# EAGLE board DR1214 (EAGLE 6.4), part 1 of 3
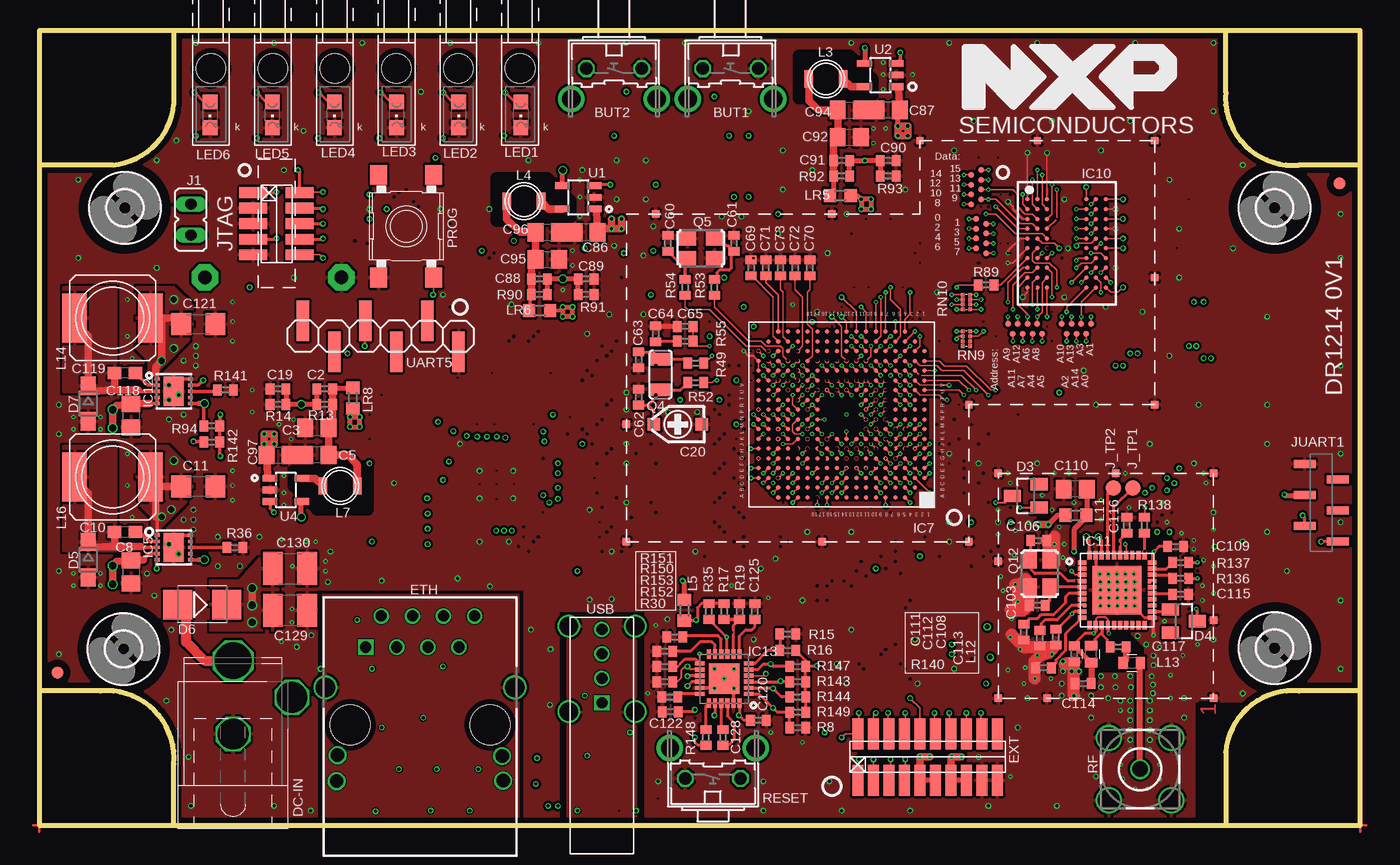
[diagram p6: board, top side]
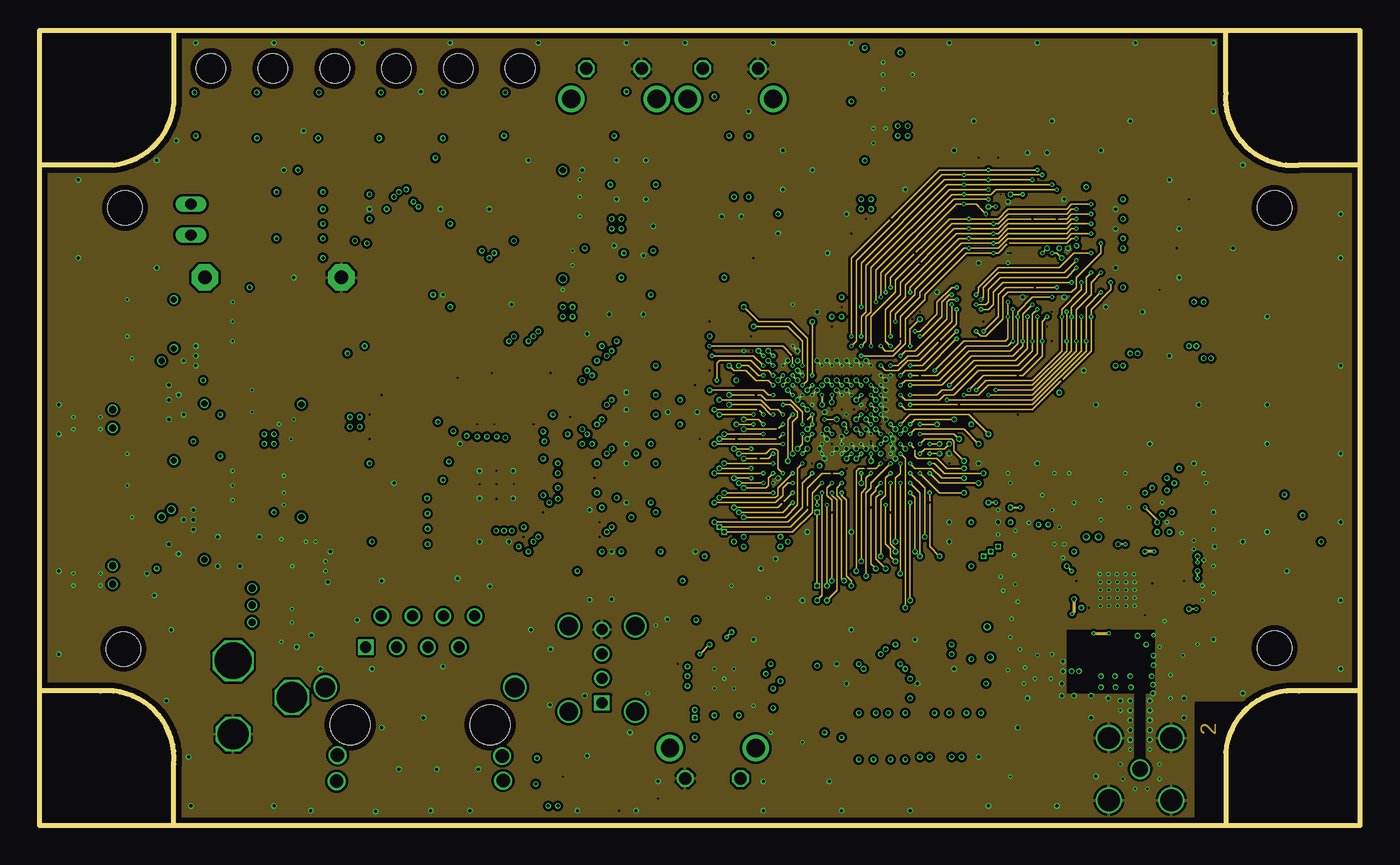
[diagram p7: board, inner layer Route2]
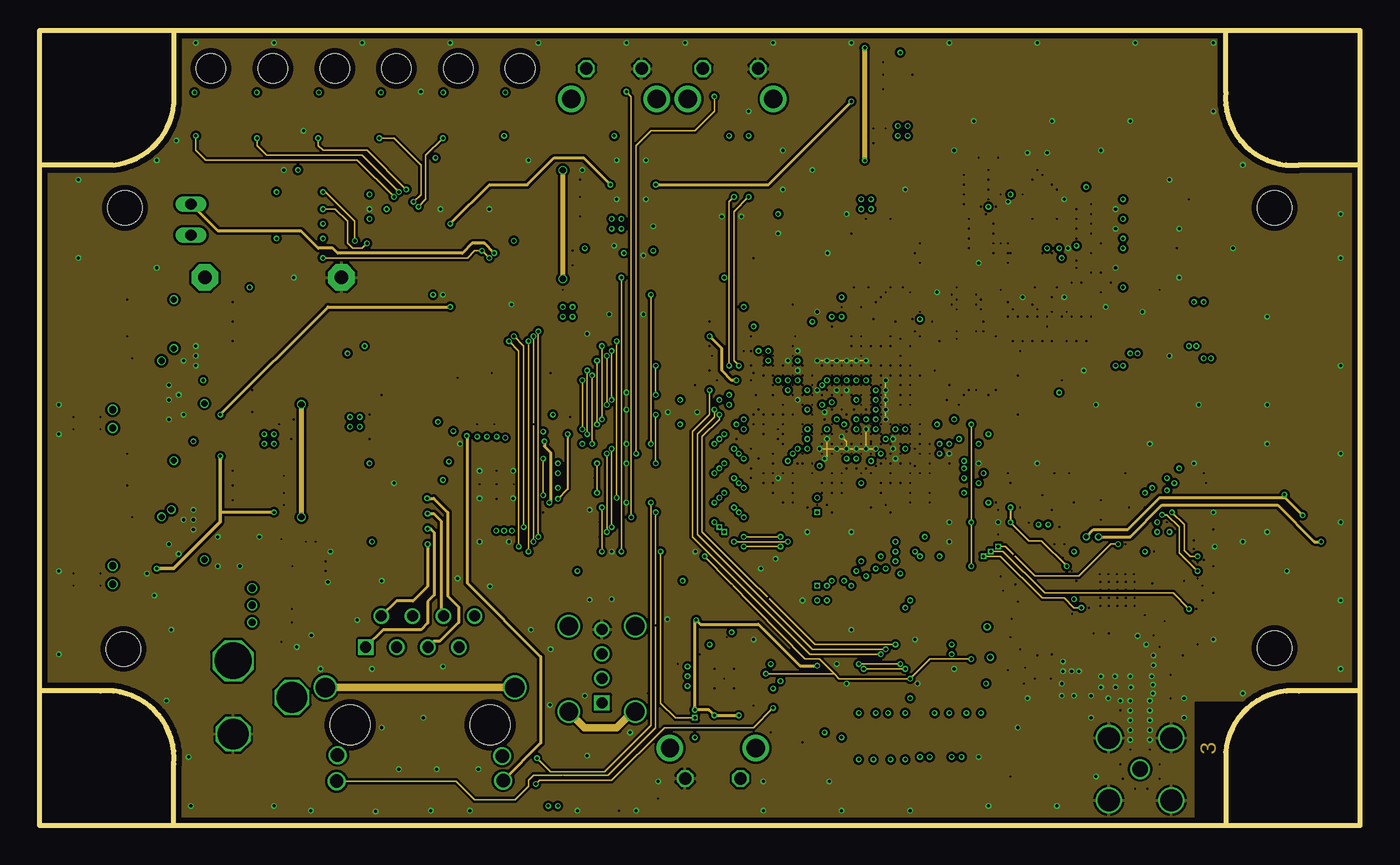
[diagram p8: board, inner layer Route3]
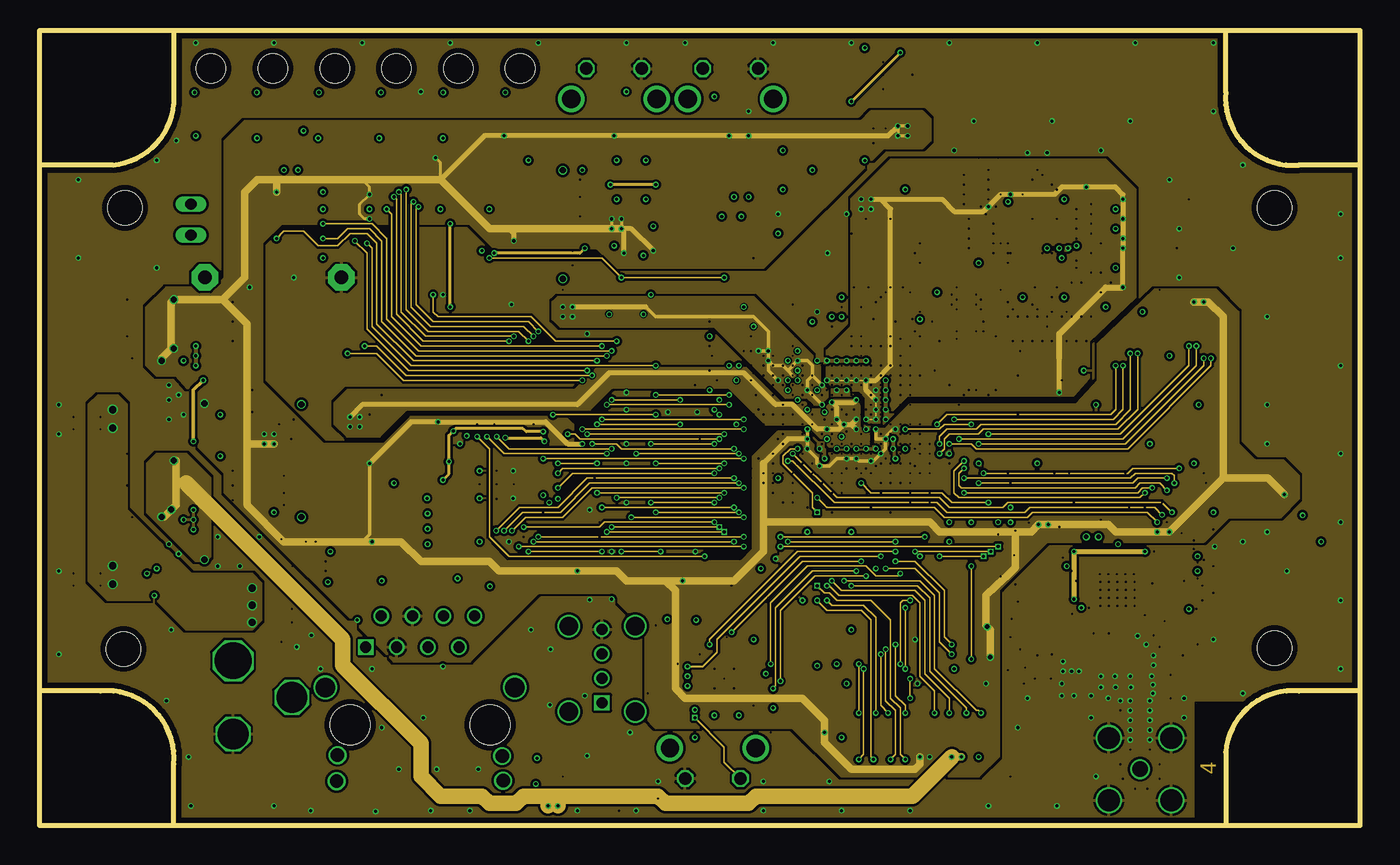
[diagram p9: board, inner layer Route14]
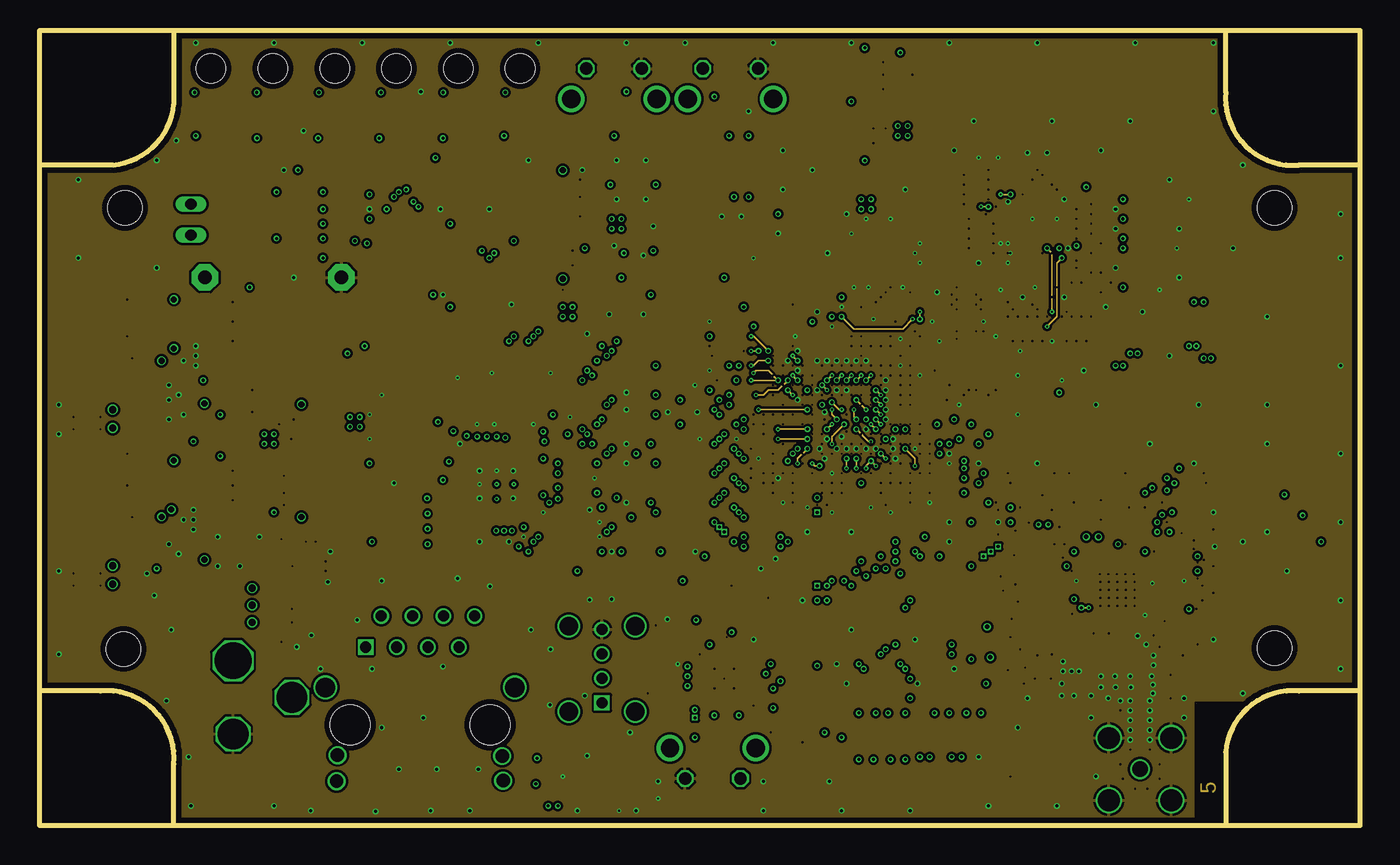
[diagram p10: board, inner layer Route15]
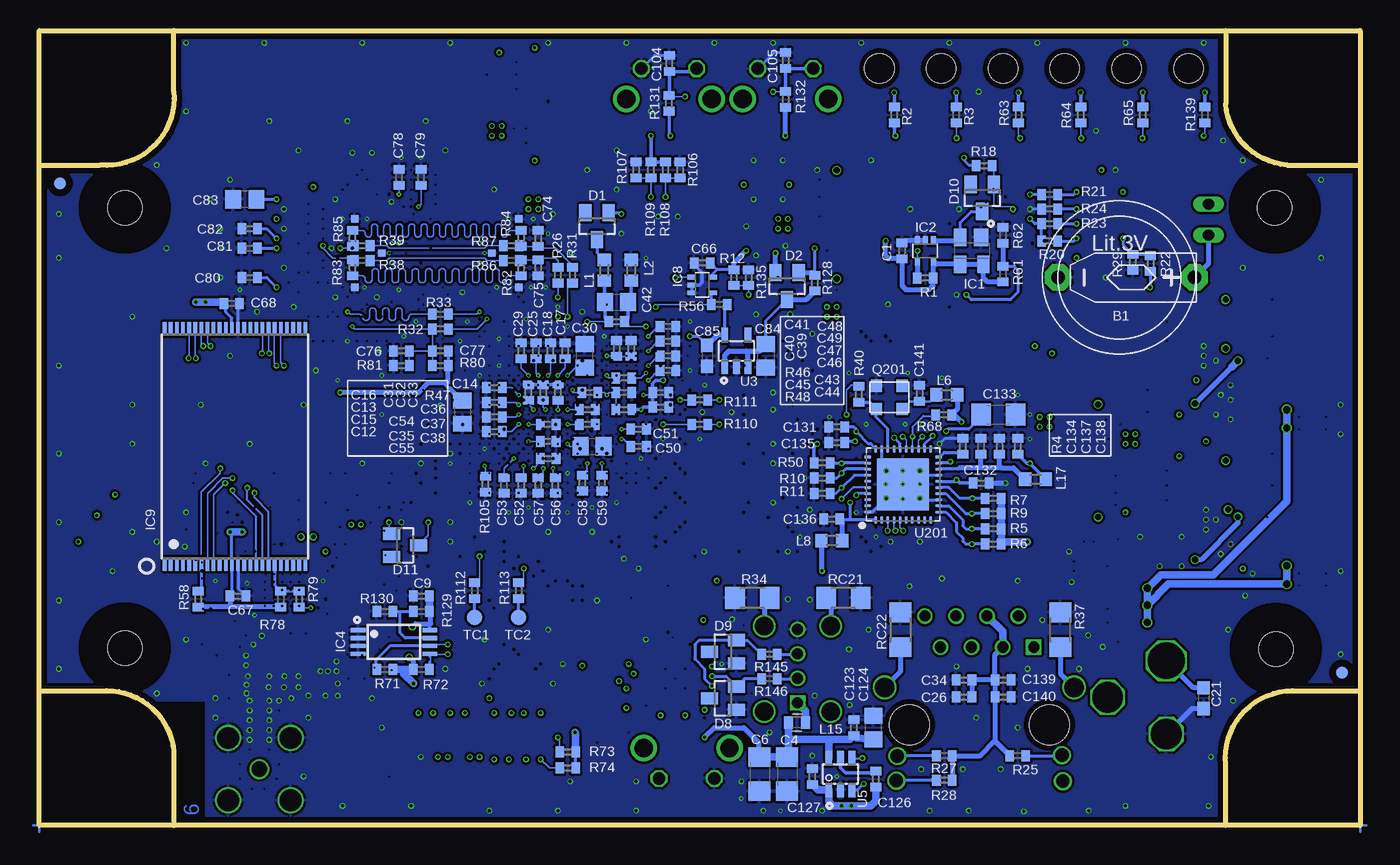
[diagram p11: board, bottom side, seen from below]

Size 108 x 65 mm. Coordinates in mm from the lower left corner, seen from the top.
Outline: 108,0 108,65
Outline: 108,65 0,65
Outline: 11,0 97,0
Outline: 97,0 108,0
Outline: 108,0 108,11
Outline: 108,11 108,54
Outline: 108,54 108,65
Outline: 108,65 97,65
Outline: 97,65 11,65
Outline: 11,65 0,65
Outline: 0,65 0,54
Outline: 0,54 0,11
Outline: 0,11 0,0 11,0
Outline: 11,0 11,5 arc100 5,11 0,11
Outline: 11,65 11,59 arc-80 6,54 0,54
Outline: 108,54 103,54 arc-100 97,60 97,65
Outline: 108,11 103,11 arc90 97,6 97,0
Copper layers ([2:1+(2*3+14*15)+16:15]): Top 0.012mm / dielectric 0.15mm / Route2 0.018mm / dielectric 0.3mm / Route3 0.018mm / dielectric 0.3mm / Route14 0.018mm / dielectric 0.3mm / Route15 0.018mm / dielectric 0.15mm / Bottom 0.012mm
Design rules "eC-TECH_pool-6-layer *": minimum track width 0.1mm, minimum drill 0.15mm, track to track 0.1mm, track to pad 0.1mm, pad to pad 0.1mm, via to via 0.1mm, smd to smd 0.1mm, copper to edge 0.45mm, drill to drill 0.3mm, minimum pad ring 0.175mm, minimum via ring 0.1mm, stop-mask expansion 0.1mm, vias tented up to drill 0.15mm, thermal gap 0.2mm
Net classes: 1 high_pow: width 1.27 mm; 2 med_pow: width 0.61 mm
tRestrict: area 37.4,49.5 to 43.4,52.9; area 20.8,25.9 to 26.8,29.3; area 62.1,59.5 to 68.1,62.9; area 58.8,26.8 to 72.4,40.4; area 85.6,12 to 90,16.9; area 80.8,44 to 82.4,51.2; area 85.6,44 to 87.2,51.2

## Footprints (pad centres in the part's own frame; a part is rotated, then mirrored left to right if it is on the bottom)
B0,5MM = smd 0.5 x 0.5: TP 0,0
CR1225H = drill 1.1 pad 2.184 octagon: + 0,6.16; - 0,-5
TACT90L = drill 1.016 octagon: 1 -2.261,-1.245; 2 2.261,-1.245 | drill 1.499 pad 2.159: 3 -3.505,1.245; 4 3.505,1.245
C0402 = smd 0.7 x 0.9: 1 -0.65,0; 2 0.65,0
C0805 = smd 1.3 x 1.5: 1 -0.95,0; 2 0.95,0
C1206 = smd 1.6 x 1.8: 1 -1.4,0; 2 1.4,0
C0603 = smd 1.1 x 1: 1 -0.85,0; 2 0.85,0
CTRIMCTZ3 = smd 1.016 x 1.016: 1 0,1.95; 2 0,-1.95
C1210 = smd 1.6 x 2.7: 1 -1.4,0; 2 1.4,0
SOT23 = smd 1 x 1.4: 1 -0.95,-1.1; 2 0.95,-1.1; 3 0,1.1
SOD323-W = smd 1.5 x 1.2: A 1.45,0; C -1.45,0
SOD128 = smd 2.4 x 2.4: A 2,0; C -2,0
DC_BIGHOLES = drill 2.5 octagon: 1 -3,0; 2 0,-4.8 | drill 3 octagon: 3 3,0
MODULARJACK8_L = drill 0.9 square: 1 -4.445,6.35 | drill 0.9: 2 -3.175,8.89; 3 -1.905,6.35; 4 -0.635,8.89; 5 0.635,6.35; 6 1.905,8.89; 7 3.175,6.35; 8 4.445,8.89 | drill 1.1: A1 -6.752,-2.491; A2 6.705,-2.561; C1 -6.828,-4.619; C2 6.781,-4.574 | drill 1.6: S1 -7.745,3.05; S2 7.745,3.05 | hole 3.25: -5.715,0; 5.715,0
127_2R20_SMT = smd 0.889 x 2.54: 1 -5.08,-1.905; 2 -5.08,1.905; 3 -3.81,-1.905; 4 -3.81,1.905; 5 -2.54,-1.905; 6 -2.54,1.905; 7 -1.27,-1.905; 8 -1.27,1.905; 9 0,-1.905; 10 0,1.905; 11 1.27,-1.905; 12 1.27,1.905; 13 2.54,-1.905; 14 2.54,1.905; 15 3.81,-1.905; 16 3.81,1.905; 17 5.08,-1.905; 18 5.08,1.905; 19 6.35,-1.905; 20 6.35,1.905
2,8 = hole 2.8: 0,0
SOT143 = smd 1.2 x 1.44: 1 -0.75,-1.1 | smd 1 x 1.44: 2 0.95,-1.1; 3 0.95,1.1; 4 -0.95,1.1
SC70-5 = smd 0.4 x 0.7: 1 -0.65,-0.85; 2 0,-0.85; 3 0.65,-0.85; 4 0.65,0.85; 5 -0.65,0.85
TSSOP8 = smd 0.35 x 1.2: 1 -0.975,-2.925; 2 -0.325,-2.925; 3 0.325,-2.925; 4 0.975,-2.925; 5 0.975,2.925; 6 0.325,2.925; 7 -0.325,2.925; 8 -0.975,2.925
DFN10-3X3 = smd 0.25 x 0.45: 1 -1,-1.35; 2 -0.5,-1.35; 3 0,-1.35; 4 0.5,-1.35; 5 1,-1.35; 6 1,1.35; 7 0.5,1.35; 8 0,1.35; 9 -0.5,1.35; 10 -1,1.35 | smd 2.38 x 1.65: EXP 0,0
SOT1048-1 = smd 0.35 x 0.35: A3 -5.184,6.779; A4 -4.387,6.779; A5 -3.589,6.779; A6 -2.792,6.779; A7 -1.994,6.779; A8 -1.196,6.779; A9 -0.399,6.779; A10 0.399,6.779; A11 1.196,6.779; A12 1.994,6.779; A13 2.791,6.779; A14 3.589,6.779; A15 4.386,6.779; A16 5.184,6.779; B2 -5.982,5.982; B3 -5.184,5.982; B4 -4.387,5.982; B5 -3.589,5.982; B6 -2.792,5.982; B7 -1.994,5.982; B8 -1.196,5.982; B9 -0.399,5.982; B10 0.399,5.982; B11 1.196,5.982; B12 1.994,5.982; B13 2.791,5.982; B14 3.589,5.982; B15 4.386,5.982; B16 5.184,5.982; B17 5.982,5.982; C1 -6.779,5.184; C2 -5.982,5.184; C3 -5.184,5.184; C4 -4.387,5.184; C5 -3.589,5.184; C6 -2.792,5.184; C7 -1.994,5.184; C8 -1.196,5.184; C9 -0.399,5.184; C10 0.399,5.184; C11 1.196,5.184; C12 1.994,5.184; C13 2.791,5.184; C14 3.589,5.184; C15 4.386,5.184; C16 5.184,5.184; C17 5.982,5.184; C18 6.779,5.184; D1 -6.779,4.387; D2 -5.982,4.387; D3 -5.184,4.387; D4 -4.387,4.387; D5 -3.589,4.387; D6 -2.792,4.387; D7 -1.994,4.387; D8 -1.196,4.387; D9 -0.399,4.387; D10 0.399,4.387; D11 1.196,4.387; D12 1.994,4.387; D13 2.791,4.387; D14 3.589,4.387; D15 4.386,4.387; D16 5.184,4.387; D17 5.982,4.387; D18 6.779,4.387; E1 -6.779,3.589; E2 -5.982,3.589; E3 -5.184,3.589; E4 -4.387,3.589; E5 -3.589,3.589; E6 -2.792,3.589; E7 -1.994,3.589; E8 -1.196,3.589; E9 -0.399,3.589; E10 0.399,3.589; E11 1.196,3.589; E12 1.994,3.589; E13 2.791,3.589; E14 3.589,3.589; E15 4.386,3.589; E16 5.184,3.589; E17 5.982,3.589; E18 6.779,3.589; F1 -6.779,2.792; F2 -5.982,2.792; F3 -5.184,2.792; F4 -4.387,2.792; F5 -3.589,2.792; F6 -2.792,2.792; F7 -1.994,2.792; F8 -1.196,2.792; F9 -0.399,2.792; F10 0.399,2.792; F11 1.196,2.792; F12 1.994,2.792; F13 2.791,2.792; F14 3.589,2.792; F15 4.386,2.792; F16 5.184,2.792; F17 5.982,2.792; F18 6.779,2.792; G1 -6.779,1.994; G2 -5.982,1.994; G3 -5.184,1.994; G4 -4.387,1.994; G5 -3.589,1.994; G6 -2.792,1.994; G7 -1.994,1.994; G8 -1.196,1.994; G9 -0.399,1.994; G10 0.399,1.994; G11 1.196,1.994; G12 1.994,1.994; G13 2.791,1.994; G14 3.589,1.994; G15 4.386,1.994; G16 5.184,1.994; G17 5.982,1.994; G18 6.779,1.994; H1 -6.779,1.196; H2 -5.982,1.196; H3 -5.184,1.196; H4 -4.387,1.196; H5 -3.589,1.196; H6 -2.792,1.196; H7 -1.994,1.196; H12 1.994,1.196; H13 2.791,1.196; H14 3.589,1.196; H15 4.386,1.196; H16 5.184,1.196; H17 5.982,1.196; H18 6.779,1.196; J1 -6.779,0.399; J2 -5.982,0.399; J3 -5.184,0.399; J4 -4.387,0.399; J5 -3.589,0.399; J6 -2.792,0.399; J7 -1.994,0.399; J12 1.994,0.399; J13 2.791,0.399; J14 3.589,0.399; J15 4.386,0.399; J16 5.184,0.399; J17 5.982,0.399; J18 6.779,0.399; K1 -6.779,-0.399; K2 -5.982,-0.399; K3 -5.184,-0.399; K4 -4.387,-0.399; K5 -3.589,-0.399; K6 -2.792,-0.399; K7 -1.994,-0.399; K12 1.994,-0.399; K13 2.791,-0.399; K14 3.589,-0.399; K15 4.386,-0.399; K16 5.184,-0.399; K17 5.982,-0.399; K18 6.779,-0.399; L1 -6.779,-1.196; L2 -5.982,-1.196; L3 -5.184,-1.196; L4 -4.387,-1.196; L5 -3.589,-1.196; L6 -2.792,-1.196; L7 -1.994,-1.196; L12 1.994,-1.196; L13 2.791,-1.196; L14 3.589,-1.196; L15 4.386,-1.196; L16 5.184,-1.196; L17 5.982,-1.196; L18 6.779,-1.196; M1 -6.779,-1.994; M2 -5.982,-1.994; M3 -5.184,-1.994; M4 -4.387,-1.994; M5 -3.589,-1.994; M6 -2.792,-1.994; M7 -1.994,-1.994; M8 -1.196,-1.994; M9 -0.399,-1.994; M10 0.399,-1.994; M11 1.196,-1.994; M12 1.994,-1.994; M13 2.791,-1.994; M14 3.589,-1.994; M15 4.386,-1.994; M16 5.184,-1.994; M17 5.982,-1.994; M18 6.779,-1.994; N1 -6.779,-2.791; N2 -5.982,-2.791; N3 -5.184,-2.791; N4 -4.387,-2.791; N5 -3.589,-2.791; N6 -2.792,-2.791; N7 -1.994,-2.791; N8 -1.196,-2.791; N9 -0.399,-2.791; N10 0.399,-2.791; N11 1.196,-2.791; N12 1.994,-2.791; N13 2.791,-2.791; N14 3.589,-2.791; N15 4.386,-2.791; N16 5.184,-2.791; N17 5.982,-2.791; N18 6.779,-2.791; P1 -6.779,-3.589; P2 -5.982,-3.589; P3 -5.184,-3.589; P4 -4.387,-3.589; P5 -3.589,-3.589; P6 -2.792,-3.589; P7 -1.994,-3.589; P8 -1.196,-3.589; P9 -0.399,-3.589; P10 0.399,-3.589; P11 1.196,-3.589; P12 1.994,-3.589; P13 2.791,-3.589; P14 3.589,-3.589; P15 4.386,-3.589; P16 5.184,-3.589; P17 5.982,-3.589; P18 6.779,-3.589; R1 -6.779,-4.386; R2 -5.982,-4.386; R3 -5.184,-4.386; R4 -4.387,-4.386; R5 -3.589,-4.386; R6 -2.792,-4.386; R7 -1.994,-4.386; R8 -1.196,-4.386; R9 -0.399,-4.386; R10 0.399,-4.386; R11 1.196,-4.386; R12 1.994,-4.386; R13 2.791,-4.386; R14 3.589,-4.386; R15 4.386,-4.386; R16 5.184,-4.386; R17 5.982,-4.386; R18 6.779,-4.386; T1 -6.779,-5.184; T2 -5.982,-5.184; T3 -5.184,-5.184; T4 -4.387,-5.184; T5 -3.589,-5.184; T6 -2.792,-5.184; T7 -1.994,-5.184; T8 -1.196,-5.184; T9 -0.399,-5.184; T10 0.399,-5.184; T11 1.196,-5.184; T12 1.994,-5.184; T13 2.791,-5.184; T14 3.589,-5.184; T15 4.386,-5.184; T16 5.184,-5.184; T17 5.982,-5.184; T18 6.779,-5.184; U2 -5.982,-5.982; U3 -5.184,-5.982; U4 -4.387,-5.982; U5 -3.589,-5.982; U6 -2.792,-5.982; U7 -1.994,-5.982; U8 -1.196,-5.982; U9 -0.399,-5.982; U10 0.399,-5.982; U11 1.196,-5.982; U12 1.994,-5.982; U13 2.791,-5.982; U14 3.589,-5.982; U15 4.386,-5.982; U16 5.184,-5.982; U17 5.982,-5.982; V3 -5.184,-6.779; V4 -4.387,-6.779; V5 -3.589,-6.779; V6 -2.792,-6.779; V7 -1.994,-6.779; V8 -1.196,-6.779; V9 -0.399,-6.779; V10 0.399,-6.779; V11 1.196,-6.779; V12 1.994,-6.779; V13 2.791,-6.779; V14 3.589,-6.779; V15 4.386,-6.779; V16 5.184,-6.779
TSOP48 = smd 1.1 x 0.3: 1 -9.625,5.75; 2 -9.625,5.25; 3 -9.625,4.75; 4 -9.625,4.25; 5 -9.625,3.75; 6 -9.625,3.25; 7 -9.625,2.75; 8 -9.625,2.25; 9 -9.625,1.75; 10 -9.625,1.25; 11 -9.625,0.75; 12 -9.625,0.25; 13 -9.625,-0.25; 14 -9.625,-0.75; 15 -9.625,-1.25; 16 -9.625,-1.75; 17 -9.625,-2.25; 18 -9.625,-2.75; 19 -9.625,-3.25; 20 -9.625,-3.75; 21 -9.625,-4.25; 22 -9.625,-4.75; 23 -9.625,-5.25; 24 -9.625,-5.75; 25 9.625,-5.75; 26 9.625,-5.25; 27 9.625,-4.75; 28 9.625,-4.25; 29 9.625,-3.75; 30 9.625,-3.25; 31 9.625,-2.75; 32 9.625,-2.25; 33 9.625,-1.75; 34 9.625,-1.25; 35 9.625,-0.75; 36 9.625,-0.25; 37 9.625,0.25; 38 9.625,0.75; 39 9.625,1.25; 40 9.625,1.75; 41 9.625,2.25; 42 9.625,2.75; 43 9.625,3.25; 44 9.625,3.75; 45 9.625,4.25; 46 9.625,4.75; 47 9.625,5.25; 48 9.625,5.75
FBGA60-6X10 = smd 0.35 x 0.35: A1 -3.2,3.6; A2 -2.4,3.6; A3 -1.6,3.6; A7 1.6,3.6; A8 2.4,3.6; A9 3.2,3.6; B1 -3.2,2.8; B2 -2.4,2.8; B3 -1.6,2.8; B7 1.6,2.8; B8 2.4,2.8; B9 3.2,2.8; C1 -3.2,2; C2 -2.4,2; C3 -1.6,2; C7 1.6,2; C8 2.4,2; C9 3.2,2; D1 -3.2,1.2; D2 -2.4,1.2; D3 -1.6,1.2; D7 1.6,1.2; D8 2.4,1.2; D9 3.2,1.2; E1 -3.2,0.4; E2 -2.4,0.4; E3 -1.6,0.4; E7 1.6,0.4; E8 2.4,0.4; E9 3.2,0.4; F1 -3.2,-0.4; F2 -2.4,-0.4; F3 -1.6,-0.4; F7 1.6,-0.4; F8 2.4,-0.4; F9 3.2,-0.4; G1 -3.2,-1.2; G2 -2.4,-1.2; G3 -1.6,-1.2; G7 1.6,-1.2; G8 2.4,-1.2; G9 3.2,-1.2; H1 -3.2,-2; H2 -2.4,-2; H3 -1.6,-2; H7 1.6,-2; H8 2.4,-2; H9 3.2,-2; J1 -3.2,-2.8; J2 -2.4,-2.8; J3 -1.6,-2.8; J7 1.6,-2.8; J8 2.4,-2.8; J9 3.2,-2.8; K1 -3.2,-3.6; K2 -2.4,-3.6; K3 -1.6,-3.6; K7 1.6,-3.6; K8 2.4,-3.6; K9 3.2,-3.6
SOT618-1 = smd 0.7 x 0.36: 1 -2.875,2.25; 2 -2.875,1.75; 3 -2.875,1.25; 4 -2.875,0.75; 5 -2.875,0.25; 6 -2.875,-0.25; 7 -2.875,-0.75; 8 -2.875,-1.25; 9 -2.875,-1.75; 10 -2.875,-2.25; 21 2.875,-2.25; 22 2.875,-1.75; 23 2.875,-1.25; 24 2.875,-0.75; 25 2.875,-0.25; 26 2.875,0.25; 27 2.875,0.75; 28 2.875,1.25; 29 2.875,1.75; 30 2.875,2.25 | smd 0.36 x 0.7: 11 -2.25,-2.875; 12 -1.75,-2.875; 13 -1.25,-2.875; 14 -0.75,-2.875; 15 -0.25,-2.875; 16 0.25,-2.875; 17 0.75,-2.875; 18 1.25,-2.875; 19 1.75,-2.875; 20 2.25,-2.875; 31 2.25,2.875; 32 1.75,2.875; 33 1.25,2.875; 34 0.75,2.875; 35 0.25,2.875; 36 -0.25,2.875; 37 -0.75,2.875; 38 -1.25,2.875; 39 -1.75,2.875; 40 -2.25,2.875 | smd 4 x 4: VSSA 0,0
HVQFN24-4X4 = smd 0.8 x 0.35: 1 -2,1.25; 2 -2,0.75; 3 -2,0.25; 4 -2,-0.25; 5 -2,-0.75; 6 -2,-1.25; 13 2,-1.25; 14 2,-0.75; 15 2,-0.25; 16 2,0.25; 17 2,0.75; 18 2,1.25 | smd 0.35 x 0.8: 7 -1.25,-2; 8 -0.75,-2; 9 -0.25,-2; 10 0.25,-2; 11 0.75,-2; 12 1.25,-2; 19 1.25,2; 20 0.75,2; 21 0.25,2; 22 -0.25,2; 23 -0.75,2; 24 -1.25,2 | smd 2.5 x 2.5: GND 0,0
JP1 = drill 0.914 long: 1 0,-1.27; 2 0,1.27
B1,27 = smd 1.27 x 1.27: TP 0,0
127_2R10_SMT = smd 0.889 x 2.286: 1 -2.54,-1.905; 2 -2.54,1.905; 3 -1.27,-1.905; 4 -1.27,1.905; 5 0,-1.905; 6 0,1.905; 7 1.27,-1.905; 8 1.27,1.905; 9 2.54,-1.905; 10 2.54,1.905
BD075-06-A-1-L-D = smd 0.65 x 1.8: 1 -3.175,-1.35; 2 -1.905,1.35; 3 -0.635,-1.35; 4 0.635,1.35; 5 1.905,-1.35; 6 3.175,1.35
R0603 = smd 1 x 1.1: 1 -0.85,0; 2 0.85,0
COIL2.8MM = smd 0.7 x 1.4: P$1 -1.4,0; P$2 1.4,0
PACKAGE0603 = smd 1 x 1.1: 1 -0.85,0; 2 0.85,0
P0603 = smd 0.762 x 1.016: 1 -0.7,0; 2 0.7,0
COIL7070 = smd 4 x 2: 1 0,3.104; 2 0,-3.104
CHIPLED_0805 = smd 1.2 x 1.2: A 0,-1.05; C 0,1.05
B3XS = smd 1.6 x 1.4: 1 -4.2,2.25; 2 4.2,2.25; 3 -4.2,-2.25; 4 4.2,-2.25
XTAL2 = smd 1 x 1.8: 1 -1.19,0; 2 1.31,0
XTAL4 = smd 1.4 x 1.15: 1 -1.6,-0.8; 2 0.6,-0.8; 3 0.6,0.8; 4 -1.6,0.8
ASE = smd 0.9 x 1: 1 -1.05,-0.95; 3 1.05,-0.95; 4 1.05,0.95; 6 -1.05,0.95
R0402 = smd 0.7 x 0.9: 1 -0.65,0; 2 0.65,0
R1206 = smd 1.6 x 1.803: 1 -1.422,0; 2 1.422,0
TACT90 = drill 1.016 octagon: 1 -2.261,0.025; 2 2.261,0.025 | drill 1.499 pad 2.159: 3 -3.505,2.515; 4 3.505,2.515
BU-SMA-V = drill 1.27: 1 0,0 | drill 1.778: 2 -2.55,2.55; 3 2.55,2.55; 4 2.55,-2.55; 5 -2.55,-2.55
EXB18V = smd 0.3 x 0.3: 1 -0.6,-0.3; 2 -0.2,-0.3; 3 0.2,-0.3; 4 0.6,-0.3; 5 0.6,0.3; 6 0.2,0.3; 7 -0.2,0.3; 8 -0.6,0.3
TP06SQ = smd 0.6 x 0.6: TP 0,0
SOT23-5 = smd 0.55 x 1.2: 1 -0.95,-1.3; 2 0,-1.3; 3 0.95,-1.3; 4 0.95,1.3; 5 -0.95,1.3
SOT23-6 = smd 0.55 x 1.2: 1 -0.95,-1.3; 2 0,-1.3; 3 0.95,-1.3; 4 0.95,1.3; 5 0,1.3; 6 -0.95,1.3
MVER_ETHERNET_LLP40 = smd 0.25 x 0.6: 1 2.25,2.9; 2 1.75,2.9; 3 1.25,2.9; 4 0.75,2.9; 5 0.25,2.9; 6 -0.25,2.9; 7 -0.75,2.9; 8 -1.25,2.9; 9 -1.75,2.9; 10 -2.25,2.9; 21 -2.25,-2.9; 22 -1.75,-2.9; 23 -1.25,-2.9; 24 -0.75,-2.9; 25 -0.25,-2.9; 26 0.25,-2.9; 27 0.75,-2.9; 28 1.25,-2.9; 29 1.75,-2.9; 30 2.25,-2.9 | smd 0.6 x 0.25: 11 -2.9,2.25; 12 -2.9,1.75; 13 -2.9,1.25; 14 -2.9,0.75; 15 -2.9,0.25; 16 -2.9,-0.25; 17 -2.9,-0.75; 18 -2.9,-1.25; 19 -2.9,-1.75; 20 -2.9,-2.25; 31 2.9,-2.25; 32 2.9,-1.75; 33 2.9,-1.25; 34 2.9,-0.75; 35 2.9,-0.25; 36 2.9,0.25; 37 2.9,0.75; 38 2.9,1.25; 39 2.9,1.75; 40 2.9,2.25 | smd 4.3 x 4.3: 41 0,0
LIGHTPIPE6 = hole 2.4: -12.64,0; -7.59,0; -2.54,0; 2.51,0; 7.56,0; 12.64,0
FIDUCIAL_1MMCIRCLE = smd 1 x 1: P$1 0,0
1X06SMD = smd 1.016 x 3.302: 1 -1.27,1.27; 2 1.27,-1.27; 3 3.81,1.27; 4 6.35,-1.27; 5 8.89,1.27; 6 11.43,-1.27
USB_A_HU = drill 0.9 square: 1 0.73,0 | drill 0.9: 2 2.73,0; 3 4.73,0; 4 6.73,0 | drill 1.5: P$5 0,2.72; P$6 0,-2.72; P$7 7,2.72; P$8 7,-2.72

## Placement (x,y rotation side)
0  TP0.5  [B0,5MM]  76.6,49.6 0 top
1  TP0.5  [B0,5MM]  77.4,49.2 0 top
2  TP0.5  [B0,5MM]  76.6,48.8 0 top
3  TP0.5  [B0,5MM]  77.4,48.4 0 top
4  TP0.5  [B0,5MM]  76.6,48 0 top
5  TP0.5  [B0,5MM]  77.4,47.6 0 top
6  TP0.5  [B0,5MM]  76.6,47.2 0 top
7  TP0.5  [B0,5MM]  77.4,46.8 0 top
8  TP0.5  [B0,5MM]  76.2,50.8 0 top
9  TP0.5  [B0,5MM]  77,51.2 0 top
10  TP0.5  [B0,5MM]  76.2,51.6 0 top
11  TP0.5  [B0,5MM]  77,52 0 top
12  TP0.5  [B0,5MM]  76.2,52.4 0 top
13  TP0.5  [B0,5MM]  77,52.8 0 top
14  TP0.5  [B0,5MM]  76.2,53.2 0 top
15  TP0.5  [B0,5MM]  77,53.6 0 top
A0  TP0.5  [B0,5MM]  85.6,40.2 0 top
A1  TP0.5  [B0,5MM]  86,41 0 top
A2  TP0.5  [B0,5MM]  84,40.2 0 top
A3  TP0.5  [B0,5MM]  85.2,41 0 top
A4  TP0.5  [B0,5MM]  81.2,40.2 0 top
A5  TP0.5  [B0,5MM]  82,40.2 0 top
A6  TP0.5  [B0,5MM]  80.8,41 0 top
A7  TP0.5  [B0,5MM]  80.4,40.2 0 top
A8  TP0.5  [B0,5MM]  81.6,41 0 top
A9  TP0.5  [B0,5MM]  79.2,41 0 top
A10  TP0.5  [B0,5MM]  83.6,41 0 top
A11  TP0.5  [B0,5MM]  79.6,40.2 0 top
A12  TP0.5  [B0,5MM]  80,41 0 top
A13  TP0.5  [B0,5MM]  84.4,41 0 top
A14  TP0.5  [B0,5MM]  84.8,40.2 0 top
B1  CR1225H  [CR1225H]  19.7,44.81 270 bottom
BUT1  MCDTSA6-5K  [TACT90L]  56.52,60.64 180 top
BUT2  MCDTSA6-5K  [TACT90L]  46.99,60.64 180 top
C1  100n  [C0402]  37.47,46.99 90 bottom
C2  12p  [C0402]  23.34,35.7 180 top
C3  4u7/X7R  [C0805]  22.7,32.52 180 top
C4  22u/X7R  [C1206]  46.85,4.2 270 bottom
C5  4u7/X7R  [C0805]  22.7,30.3 180 top
C6  22u/X7R  [C1206]  49.1,4.2 270 bottom
C8  4u7/X7R  [C0805]  7.5,20.73 270 top
C9  100n  [C0402]  76.75,18.75 0 bottom
C10  470n  [C0603]  7,24 180 top
C11  22u/X7R  [C1206]  13,27.73 0 top
C12  10n  [C0402]  70.8,32.2 180 bottom
C13  100n  [C0402]  70.8,34.6 180 bottom
C14  10u/X7R  [C0805]  73.4,33.8 270 bottom
C15  10n  [C0402]  70.8,33.4 180 bottom
C16  100n  [C0402]  70.8,35.8 180 bottom
C17  10n  [C0402]  65,38.8 90 bottom
C18  10n  [C0402]  66.2,38.8 90 bottom
C19  na  [C0402]  19.52,35.7 180 top
C20  5-20p  [CTRIMCTZ3]  52.2,32.8 90 top
C21  10n/NP0  [C0603]  12.8,10.4 270 bottom
C25  100n  [C0402]  67.4,38.8 90 bottom
C26  100n  [C0402]  32.4,10.5 180 bottom
C29  100n  [C0402]  68.6,38.8 90 bottom
C30  10u/X7R  [C0805]  63.4,38.4 90 bottom
C31  10n  [C0402]  68,35.4 90 bottom
C32  10n  [C0402]  66.8,35.4 90 bottom
C33  10n  [C0402]  65.6,35.4 90 bottom
C34  100n  [C0402]  32.4,11.9 180 bottom
C35  100n  [C0402]  66.4,31.4 0 bottom
C36  100n  [C0402]  63.2,34 0 bottom
C37  100n  [C0402]  63.2,32.8 0 bottom
C38  10u/X7R  [C0805]  62.8,31 0 bottom
C39  10n  [C0402]  59.6,39 90 bottom
C40  100n  [C0402]  60.8,39 90 bottom
C41  10n  [C0402]  60.8,41.2 0 bottom
C42  10u/X7R  [C0805]  60.8,42.8 0 bottom
C43  100n  [C0402]  57.2,35.4 0 bottom
C44  100n  [C0402]  57.2,34.2 0 bottom
C45  100n  [C0402]  60.2,35.4 0 bottom
C46  100n  [C0402]  56.6,37.2 0 bottom
C47  100n  [C0402]  56.6,38.4 0 bottom
C48  100n  [C0402]  56.6,40.8 0 bottom
C49  100n  [C0402]  56.6,39.6 0 bottom
C50  10n  [C0402]  59,31 0 bottom
C51  100n  [C0402]  59,32.4 0 bottom
C52  10n  [C0402]  68.6,27.8 270 bottom
C53  100n  [C0402]  70,27.8 270 bottom
C54  10n  [C0402]  66.4,32.8 0 bottom
C55  100n  [C0402]  66.4,30 0 bottom
C56  10n  [C0402]  65.8,27.8 270 bottom
C57  100n  [C0402]  67.2,27.8 270 bottom
C58  10n  [C0402]  63.6,28 270 bottom
C59  100n  [C0402]  62,28 270 bottom
C60  22p  [C0402]  51.4,47.6 270 top
C61  22p  [C0402]  56.8,47.6 270 top
C62  22p  [C0402]  49,35.03 270 top
C63  22p  [C0402]  49,38.07 90 top
C64  3n9  [C0402]  50.4,40.2 270 top
C65  150p  [C0402]  52.8,40.8 0 top
C66  100n  [C0402]  53.8,46 180 bottom
C67  10n  [C0402]  91.75,18.75 0 bottom
C68  100n  [C0402]  92.27,42.69 0 bottom
C69  1n  [C0402]  58.2,45.6 90 top
C70  1n  [C0402]  63,45.6 90 top
C71  1n  [C0402]  59.4,45.6 90 top
C72  1n  [C0402]  61.8,45.6 90 top
C73  1n  [C0402]  60.6,45.6 90 top
C74  na  [C0402]  67.2,48 90 bottom
C75  na  [C0402]  67.2,45.6 270 bottom
C76  na  [C0402]  78.4,38.8 180 bottom
C77  na  [C0402]  75.2,38.8 180 bottom
C78  10n  [C0402]  78.6,53 90 bottom
C79  10n  [C0402]  76.8,53 90 bottom
C80  100n  [C0402]  90.8,44.8 180 bottom
C81  100n  [C0402]  90.8,47.2 180 bottom
C82  100n  [C0402]  90.8,48.8 180 bottom
C83  10u/X7R  [C0805]  91.2,51.2 180 bottom
C84  4u7/X7R  [C0805]  48.6,38.4 270 bottom
C85  470n/X7R  [C0603]  53.4,38.4 270 bottom
C86  4u7/X7R  [C0805]  44.7,48.5 180 top
C87  4u7/X7R  [C0805]  69.41,58.5 180 top
C88  na  [C0402]  40.9,44.69 0 top
C89  na  [C0402]  44.7,44.69 0 top
C90  na  [C0402]  69.41,54.38 0 top
C91  na  [C0402]  65.59,54.38 0 top
C92  4u7/X7R  [C0805]  66.23,56.28 0 top
C94  4u7/X7R  [C0805]  66.23,58.5 0 top
C95  4u7/X7R  [C0805]  41.53,46.28 0 top
C96  4u7/X7R  [C0805]  41.53,48.5 0 top
C97  4u7/X7R  [C0805]  19.52,30.3 0 top
C103  15p  [C0402]  81.6,18 0 top
C104  22n  [C0402]  56.48,62.3 90 bottom
C105  22n  [C0402]  46.99,62.55 90 bottom
C106  15p  [C0402]  81.7,23.3 180 top
C108  100n/X7R  [C0402]  83.1,15.4 270 top
C109  100n/X7R  [C0402]  92.9,22.8 0 top
C110  10u/X7R  [C0805]  84.7,27.5 180 top
C111  100n/X7R  [C0402]  80.5,15.8 270 top
C112  10n/X7R  [C0402]  81.8,15.3 270 top
C113  47p/NPO  [C0402]  84.62,14.03 270 top
C114  100n/X7R  [C0402]  85.33,11.61 180 top
C115  100n/X7R  [C0402]  93.3,18.9 0 top
C116  100n/X7R  [C0402]  88.9,24.55 90 top
C117  47p/NPO  [C0402]  88.2,14.6 180 top
C118  4u7/X7R  [C0805]  7.5,33.5 270 top
C119  470n  [C0603]  7,37 180 top
C120  100n  [C0402]  58.8,8.6 0 top
C121  22u/X7R  [C1206]  13,41 0 top
C122  100n  [C0402]  51.6,9.3 180 top
C123  100n  [C0402]  41.4,8 90 bottom
C124  4u7/X7R  [C0805]  39.8,8 90 bottom
C125  1u  [C0402]  58.5,17.5 90 top
C126  1n  [C0402]  39.6,3.8 270 bottom
C127  100n  [C0402]  44.8,4 90 bottom
C128  220n  [C0402]  55.9,7.2 270 top
C129  47u/16v  [C1210]  20.5,17.6 0 top
C130  47u/16v  [C1210]  20.5,21 0 top
C131  100n  [C0402]  42.8,32.6 180 bottom
C132  100n  [C0402]  31,28 0 bottom
C133  10u/tantalium  [C1206]  29.59,33.6 0 bottom
C134  1u  [C0402]  31,31 90 bottom
C135  1u  [C0402]  42.8,31.3 180 bottom
C136  100n  [C0402]  43.2,25.05 180 bottom
C137  100n  [C0402]  29.5,31 90 bottom
C138  2u2  [C0402]  28,31 90 bottom
C139  100n  [C0402]  29.2,11.9 0 bottom
C140  100n  [C0402]  29.2,10.5 0 bottom
C141  100n  [C0402]  36.02,35.33 90 bottom
D1  BAT754  [SOT23]  62.4,49 180 bottom
D2  BAT54C  [SOT23]  46.86,44.11 180 bottom
D3  BAT754  [SOT23]  80.65,26.95 90 top
D4  BAT754  [SOT23]  93.58,16.71 270 top
D5  PMEG2010AEJ  [SOD323-W]  4,21.73 270 top
D6  PMEG3020EP  [SOD128]  13.32,18.07 180 top
D7  PMEG2010AEJ  [SOD323-W]  4,34.5 270 top
D8  MMBZ9V1AL  [SOT23]  52.1,10.4 90 bottom
D9  MMBZ9V1AL  [SOT23]  52.1,14.2 90 bottom
D10  BAT754  [SOT23]  30.9,51.32 180 bottom
D11  BAT754  [SOT23]  78.1,22.9 270 bottom
DC-IN  DC10B  [DC_BIGHOLES]  15.85,10.47 90 top
ETH  TE CONNECTIVITY - 5-6605758-1  [MODULARJACK8_L]  31.14,8.23 0 top
EXT  M50-3601042  [127_2R20_SMT]  72,5.6 0 top
FM1  CROSSHAIR8MIL  [CROSSHAIR_8MIL]  108,0 0 top
FM2  CROSSHAIR8MIL  [CROSSHAIR_8MIL]  0,0 0 top
FM3  CROSSHAIR8MIL  [CROSSHAIR_8MIL]  108,0 0 bottom
FM4  CROSSHAIR8MIL  [CROSSHAIR_8MIL]  0,0 0 bottom
H1  MOUNT-HOLE2.8  [2,8]  7,50.5 0 top
H2  MOUNT-HOLE2.8  [2,8]  6.89,14.43 0 top
H3  MOUNT-HOLE2.8  [2,8]  101,50.5 0 top
H4  MOUNT-HOLE2.8  [2,8]  101,14.5 0 top
IC1  CAT811S  [SOT143]  31.75,46.99 180 bottom
IC2  74LVC1G125GW  [SC70-5]  35.56,46.99 180 bottom
IC4  24LC256-I/ST  [TSSOP8]  79,15 270 bottom
IC5  LT3971EDD-5  [DFN10-3X3]  11,22.73 270 top
IC7  LPC32X0  [SOT1048-1]  65.6,33.6 180 top
IC8  74LVC1G125GW  [SC70-5]  53.8,44.2 270 bottom
IC9  NAND01GW3B2CN6E  [TSOP48]  92,31 90 bottom
IC10  H5MS5162EFR  [FBGA60-6X10]  84,47.6 0 top
IC11  JN516X  [SOT618-1]  88.12,19.24 0 top
IC12  LT3971EDD-3.3  [DFN10-3X3]  11,35.5 270 top
IC13  STOTG04E  [HVQFN24-4X4]  56,12 180 top
J1  BAT_EN (nc)  [JP1]  12.4,49.55 180 top
J_TP1  TPB1,27  [B1,27]  89.4,27.6 0 top
J_TP2  TPB1,27  [B1,27]  87.8,27.6 0 top
JTAG  M50-3600542  [127_2R10_SMT]  19.4,49.2 270 top
JUART1  BD075-06-A-1-L-D  [BD075-06-A-1-L-D]  104.8,26.4 90 top
L1  BLM18AG221SN1D  [R0603]  61.8,45.4 270 bottom
L2  BLM18AG221SN1D  [R0603]  59.6,45.4 270 bottom
L3  VLF3010AT-2R2M1R0  [COIL2.8MM]  64.33,61.04 180 top
L4  VLF3010AT-2R2M1R0  [COIL2.8MM]  39.62,51.04 180 top
L5  BLM18AG601S  [PACKAGE0603]  52.75,17.6 270 top
L6  BLM18AG601S  [PACKAGE0603]  33.8,35.2 0 bottom
L7  VLF3010AT-2R2M1R0  [COIL2.8MM]  24.61,27.76 0 top
L8  BLM18AG601S  [PACKAGE0603]  43.2,23.3 180 bottom
L11  BLM18AG221SN1D  [R0603]  84.75,25.35 180 top
L12  3n9H, LQP15MN3N9B02  [P0603]  86,14 90 top
L13  5n1H, LQP15MN5N1B02  [P0603]  89.32,13.29 0 top
L14  SLF7045, 3.3uH  [COIL7070]  6,41.5 90 top
L15  BK1608HS220  [P0603]  46.05,8.4 180 bottom
L16  SLF7045, 3.3uH  [COIL7070]  6,28.5 90 top
L17  BLM18AG601S  [PACKAGE0603]  26.55,28.3 0 bottom
LED1  OVS-0803(B)  [CHIPLED_0805]  39.37,58.1 180 top
LED2  OVS-0806(Y)  [CHIPLED_0805]  34.29,58.1 180 top
LED3  OVS-0808(R)  [CHIPLED_0805]  29.21,58.1 180 top
LED4  OVS-0804(G)  [CHIPLED_0805]  24.13,58.1 180 top
LED5  OVS-0806(Y)  [CHIPLED_0805]  19.05,58.1 180 top
LED6  OVS-0808(R)  [CHIPLED_0805]  13.97,58.1 180 top
LR5  0E  [R0603]  65.5,51.5 0 top
LR6  0E  [R0603]  40.91,42.1 0 top
LR8  0E  [R0603]  25.63,34.94 270 top
PROG  B3S1000  [B3XS]  30,49 270 top
Q4  32.768kHz  [XTAL2]  50.8,36.93 270 top
Q5  12MHz  [XTAL4]  53.6,47.2 180 top
Q12  32MHz  [XTAL4]  81.8,20.1 270 top
Q201  ASEMPC-50.000MHZ-LR-T  [ASE]  38.5,35 180 bottom
R1  33k  [R0402]  35.56,44.77 0 bottom
R2  150E  [R0402]  38.1,58.1 270 bottom
R3  470E  [R0402]  33.02,58.1 270 bottom
R4  4k87/1%  [R0402]  32.5,31 90 bottom
R5  50E  [R0402]  30,24.25 0 bottom
R6  50E  [R0402]  30,23 0 bottom
R7  50E  [R0402]  30,26.75 0 bottom
R8  na  [R0402]  62,8 180 top
R9  50E  [R0402]  30,25.5 0 bottom
R10  na  [R0402]  44,28.4 180 bottom
R11  na  [R0402]  44,27.15 180 bottom
R12  na (0E for boundary scan)  [R0402]  51.2,44.8 270 bottom
R13  300k  [R0402]  23.34,34.42 0 top
R14  180k  [R0402]  19.52,34.42 0 top
R15  na  [R0402]  61.2,15.65 180 top
R16  0E  [R0402]  61.2,14.3 0 top
R17  0E  [R0402]  56,17.5 90 top
R18  10k  [R0402]  30.75,53.95 180 bottom
R19  na  [R0402]  57.25,17.5 270 top
R20  10k  [R0402]  25.4,47.8 180 bottom
R21  10k  [R0402]  25.4,51.6 180 bottom
R22  10k  [R0402]  17.15,45.95 270 bottom
R23  10k  [R0402]  25.4,49.2 180 bottom
R24  10k  [R0402]  25.4,50.4 0 bottom
R25  120E  [R0402]  28,5.7 0 bottom
R26  0E  [R0402]  65.6,45 90 bottom
R27  120E  [R0402]  34,5.7 180 bottom
R28  2k2  [R0402]  34,3.7 180 bottom
R29  na  [R0402]  18.6,46.05 90 bottom
R30  1k  [R0402]  51.55,10.5 0 top
R31  0E  [R0402]  64.4,45 90 bottom
R32  na  [R0402]  75.2,40.6 180 bottom
R33  22E  [R0402]  75.2,41.8 180 bottom
R34  0E  [R1206]  49.7,18.6 0 bottom
R35  100k  [R0402]  54.75,17.5 90 top
R36  14k  [R0402]  16,22.73 180 top
R37  0E  [R1206]  24.5,16 270 bottom
R38  na  [R0402]  81.6,46.2 180 bottom
R39  na  [R0402]  81.6,47.4 180 bottom
R40  22E  [R0402]  41,35.25 270 bottom
R46  0E  [R0402]  60.2,36.6 0 bottom
R47  na  [R0402]  63,35.4 180 bottom
R48  0E  [R0402]  60.2,34 0 bottom
R49  0E  [R0402]  53.67,37.8 0 top
R50  2k2  [R0402]  44,29.65 0 bottom
R52  0E  [R0402]  53.67,36.2 0 top
R53  0E  [R0402]  55.2,44 270 top
R54  0E  [R0402]  52.8,44 270 top
R55  120k  [R0402]  52.8,39.6 0 top
R56  10k  [R0402]  52.4,42.6 0 bottom
R58  2k2  [R0402]  95,18.5 270 bottom
R61  10k  [R0402]  29.21,45.09 270 bottom
R62  na  [R0402]  29.21,48.26 270 bottom
R63  1k  [R0402]  27.94,58.1 270 bottom
R64  560E  [R0402]  22.86,58.1 270 bottom
R65  470E  [R0402]  17.78,58.1 270 bottom
R68  1k5  [R0402]  34.07,33.57 180 bottom
R71  3k3  [R0402]  79.75,12.75 0 bottom
R72  3k3  [R0402]  76.75,12.75 180 bottom
R73  3k3  [R0402]  64.8,6 0 bottom
R74  3k3  [R0402]  64.8,4.7 0 bottom
R78  33k  [R0402]  88.25,18.5 270 bottom
R79  0E  [R0402]  86.75,18.5 90 bottom
R80  4k7  [R0402]  75.2,37.6 0 bottom
R81  4k7  [R0402]  78.4,37.6 0 bottom
R82  0E  [R0402]  68.6,45.6 90 bottom
R83  22E  [R0402]  82.4,45.6 90 bottom
R84  0E  [R0402]  68.6,48 270 bottom
R85  22E  [R0402]  82.4,48 270 bottom
R86  na  [R0402]  69.4,46.2 180 bottom
R87  na  [R0402]  69.4,47.4 180 bottom
R89  0E  [R0402]  77.4,44.2 0 top
R90  0E  [R0402]  40.9,43.42 180 top
R91  na  [R0402]  44.7,43.42 180 top
R92  0E  [R0402]  65.59,53.1 180 top
R93  na  [R0402]  69.41,53.1 180 top
R94  100k  [R0402]  14.1,32.67 180 top
R105  33k  [R0402]  71.53,27.91 90 bottom
R106  33k  [R0402]  55.6,53.6 270 bottom
R107  na  [R0402]  59.2,53.6 270 bottom
R108  na  [R0402]  56.8,53.6 90 bottom
R109  33k  [R0402]  58,53.6 90 bottom
R110  22E  [R0402]  54,32.8 0 bottom
R111  22E  [R0402]  54,34.8 0 bottom
R112  22E  [R0402]  72.4,19.2 270 bottom
R113  22E  [R0402]  68.8,19.2 270 bottom
R128  na  [R0402]  44.6,44.35 270 bottom
R129  na  [R0402]  76.75,17.5 0 bottom
R130  10k  [R0402]  79.75,17.5 0 bottom
R131  10k  [R0402]  56.52,59.05 270 bottom
R132  10k  [R0402]  46.99,59.37 270 bottom
R135  10k  [R0402]  50,44.8 270 bottom
R136  100E  [R0402]  93.3,20.2 180 top
R137  100E  [R0402]  93.3,21.5 180 top
R138  100E  [R0402]  90.35,24.55 270 top
R139  1k  [R0402]  12.7,58.1 270 bottom
R140  43k, 1%  [R0402]  82.1,12.9 180 top
R141  14k  [R0402]  15.21,35.61 180 top
R142  na  [R0402]  14.1,31.34 0 top
R143  2k2  [R0402]  62,11.75 0 top
R144  2k2  [R0402]  62,10.5 0 top
R145  20E  [R0402]  48.3,14 180 bottom
R146  20E  [R0402]  48.3,12 180 bottom
R147  10k  [R0402]  62,13 0 top
R148  1k  [R0402]  54.5,7.2 90 top
R149  100k  [R0402]  62,9.25 0 top
R150  na  [R0402]  51.15,14.25 0 top
R151  na  [R0402]  51.95,15.4 0 top
R152  47k  [R0402]  51.15,11.75 0 top
R153  47k  [R0402]  51.15,13 0 top
RC21  0E  [R1206]  42.25,18.6 0 bottom
RC22  0E  [R1206]  37.6,16 90 bottom
RESET  MCDTSA6-2K  [TACT90]  55.07,3.81 0 top
RF  nc  [BU-SMA-V]  90,4.6 0 top
RN9  22E  [EXB18V]  75.8,39.8 270 top
RN10  22E  [EXB18V]  75.8,42.8 270 top
SP1  TPTP06SQ  [TP06SQ]  78.4,28.8 0 top
SP2  TPTP06SQ  [TP06SQ]  96,28.8 0 top
SP3  TPTP06SQ  [TP06SQ]  96,10.4 0 top
SP4  TPTP06SQ  [TP06SQ]  78.4,10.4 0 top
SP5  TPTP06SQ  [TP06SQ]  82.4,10.4 0 top
SP6  TPTP06SQ  [TP06SQ]  78.4,21.6 0 top
SP7  TPTP06SQ  [TP06SQ]  88,28.8 0 top
SP8  TPTP06SQ  [TP06SQ]  96,16.8 0 top
SP9  TPTP06SQ  [TP06SQ]  48,23.2 0 top
SP10  TPTP06SQ  [TP06SQ]  64,23.2 0 top
SP11  TPTP06SQ  [TP06SQ]  76,23.2 0 top
SP12  TPTP06SQ  [TP06SQ]  76,34.4 0 top
SP13  TPTP06SQ  [TP06SQ]  91.2,34.4 0 top
SP14  TPTP06SQ  [TP06SQ]  91.2,56 0 top
SP15  TPTP06SQ  [TP06SQ]  72,56 0 top
SP16  TPTP06SQ  [TP06SQ]  64.8,50 0 top
SP17  TPTP06SQ  [TP06SQ]  50.4,50 0 top
SP18  TPTP06SQ  [TP06SQ]  48,32.8 0 top
SP19  TPTP06SQ  [TP06SQ]  91.2,44.8 0 top
SP20  TPTP06SQ  [TP06SQ]  81.6,56 0 top
SP21  TPTP06SQ  [TP06SQ]  68.8,49.6 270 bottom
SP22  TPTP06SQ  [TP06SQ]  68.8,44 270 bottom
SP23  TPTP06SQ  [TP06SQ]  71,46.8 270 bottom
SP24  TPTP06SQ  [TP06SQ]  80,46.8 270 bottom
SP25  TPTP06SQ  [TP06SQ]  82.2,44 270 bottom
SP26  TPTP06SQ  [TP06SQ]  82.2,49.6 270 bottom
TC1  TPB1,27  [B1,27]  72.4,17 180 bottom
TC2  TPB1,27  [B1,27]  68.8,17 180 bottom
U1  LM3671MF-1.2  [SOT23-5]  44.07,51.36 90 top
U2  LM3671MF-1.8  [SOT23-5]  68.77,61.36 90 top
U3  MIC5232-1.2YD5  [SOT23-5]  51,38.8 0 bottom
U4  LM3671MF-ADJ  [SOT23-5]  20.16,27.44 270 top
U5  MIC2005A-2YM6  [SOT23-6]  42.5,4.2 0 bottom
U201  DP83848-2MSQ  [MVER_ETHERNET_LLP40]  37.37,27.88 180 bottom
U$1  LIGHTPIPE6  [LIGHTPIPE6]  26.67,61.91 180 top
U$3  FICUDIAL_1MM-1  [FIDUCIAL_1MMCIRCLE]  106.3,52.5 0 bottom
U$4  FICUDIAL_1MM-1  [FIDUCIAL_1MMCIRCLE]  1.5,12.5 0 bottom
U$5  FICUDIAL_1MM-1  [FIDUCIAL_1MMCIRCLE]  106.3,52.5 0 top
U$6  FICUDIAL_1MM-1  [FIDUCIAL_1MMCIRCLE]  1.5,12.5 0 top
UART5  [1X06SMD]  33,40 180 top
USB  [USB_A_HU]  46,9.3 90 top

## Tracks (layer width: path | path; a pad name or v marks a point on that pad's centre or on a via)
!CAS  (via drill 0.15 layers 1-2)
  Top 0.127: RN10.6 v76.6,42.6 | v84.8,45.6 85.2,46 86,46 IC10.G8
  Route2 0.127: v84.8,45.6 84,44.8 78.6,44.8 77.6,43.8 77.6,42.8 77.4,42.6 v76.6,42.6
!DDR_CLK  (via drill 0.15 layers 1-2, 0.15 layers 15-16, 0.25 layers 2-15)
  Top 0.127: v82.8,46.8 IC10.G3
  Route2 0.127: v82.8,46.8 83.2,46.8 v83.6,46.4
  Route15 0.127: v83.6,46.4 83.2,46 83.2,41.6 v82.4,40.8
  Bottom 0.127: R80.1 C77.2 | C77.2 R32.2 82.2,40.6 v82.4,40.8 | C77.2 C76.1 R81.2
!EMC_CLK  (via drill 0.15 layers 15-16, 0.25)
  Top 0.127: IC7.V9 66,41.2 v65.6,41.6
  Route15 0.127: v65.6,41.6 66.6,40.6 70.6,40.6 v71.4,41.4
  Bottom 0.127: R32.1 72.2,40.6 v71.4,41.4
!RAS  (via drill 0.15 layers 1-2)
  Top 0.127: RN10.8 v76.6,43.4 | v86,46.8 86.8,46.8 IC10.G9
  Route2 0.127: v76.6,43.4 76.8,43.6 76.8,44 78.4,45.6 83.4,45.6 84.6,46.8 v86,46.8
!RESET_IN  (via drill 0.25, 0.25 layers 2-15)
  Top 0.127: JTAG.10 22.94,46.66 v23.2,46.4
  Route3 0.127: v23.2,46.4 35,46.4 35.6,47 v36.2,47 v36.8,46.4 | v47.6,44.8 v47.6,22.4 | v50.8,22.4 50.8,10 52,8.8 v53.6,8.8
  Route14 0.127: v36.8,46.4 46,46.4 v47.6,44.8 v56,44.8 | v47.6,22.4 v50.8,22.4 | v53.6,8.8 56,6.4 56,5.17 RESET.2
  Bottom 0.127: v36.2,47 IC2.4 | IC8.1 55.95,44.85 v56,44.8
  Bottom 0.406: IC2.4 R1.1
!SYS_RESET  (via drill 0.15 layers 1-2, 0.25, 0.25 layers 2-15, 0.25 pad 0.1)
  Top 0.127: IC7.G4 70.01,31.61 v70.4,32 | EXT.10 72,9.6 v71.2,10.4 | IC13.4 59.25,12.25 v59.4,12.4
  Route2 0.127: v70.4,32 v70.8,32.4
  Route3 0.127: v54.4,22 62.6,13.6 63.8,13.6 65,12.4 | 65,12.4 v59.4,12.4 | v76.2,21.2 v76.2,24.78 v76.2,32.8 | v76.2,13.6 72.8,13.6 v71.2,12 65.4,12 65,12.4
  Route14 0.127: v35.8,31.8 36.8,30.8 36.8,23.6 38.4,22 v54.4,22 | v76.2,13.6 v76.2,21.2 | v70.8,32.4 73.6,32.4 74,32.8 v76.2,32.8 | v71.2,10.4 v71.2,12
  Bottom 0.127: U201.23 36.12,31.48 v35.8,31.8 | v76.2,24.78 76.2,23.7 D11.3
!USB_ATX_INT  (via drill 0.15 pad 0.1 layers 1-2, 0.25, 0.25 layers 2-15)
  Top 0.127: IC7.C4 v70.4,28
  Top 0.254: IC13.5 58.75,12.75 59.2,13.2 v59.8,13.2 60,13 R147.1
  Route2 0.127: v70.4,28 v70.4,20.6
  Route14 0.127: v70.4,20.6 70.2,20.4 68.4,20.4 67.6,21.2 62.8,21.2 59.8,18.2 v59.8,13.2
!USB_OE_TP  (via drill 0.15 layers 1-2, 0.25 layers 2-15)
  Top 0.127: IC7.D6 68.39,29.19 v68,28.8 | 56.2,14.05 IC13.9
  Top 0.254: 56.2,14.05 v56.2,15.4 R35.1
  Route2 0.127: v56.6,15.8 v56.2,15.4 | v68,28.8 67.6,28.4 67.6,27.6 67.2,27.2 v67.2,21.6
  Route14 0.127: v67.2,21.6 62.4,21.6 v56.6,15.8
!WR  (via drill 0.15 layers 1-2)
  Top 0.127: RN10.7 v77,43 | v84.8,46.2 85,46.4 IC10.G7
  Route2 0.127: v77,43 77.2,43.2 77.2,44 78.4,45.2 83.8,45.2 v84.8,46.2
ABUS0  (via drill 0.15 layers 1-2)
  Top 0.127: IC7.L3 70.8,34.8 v71.2,34.4 | IC10.J8 86.8,44.4 v86.8,43.6 | A0.TP v85.6,39.6
  Route2 0.127: v71.2,34.4 81.2,34.4 85.6,38.8 v85.6,39.6 85.6,42.4 v86.8,43.6
ABUS1  (via drill 0.15 layers 1-2)
  Top 0.127: IC7.L4 70,34.8 v70.4,34.4 | IC10.J9 v87.6,44.4 | A1.TP v86,41.6
  Route2 0.127: v70.4,34.4 70.8,34 81.2,34 86,38.8 v86,41.6 86,42.2 87.6,43.8 v87.6,44.4
ABUS2  (via drill 0.15 layers 1-2)
  Top 0.127: IC7.M1 75.21,35.59 v75.6,35.2 | IC10.K7 84,42.4 v84,42 | v84,39.6 A2.TP
  Route2 0.127: v84,42 v84,39.6 84,38.8 81.2,36 77.6,36 76.8,35.2 v75.6,35.2
ABUS3  (via drill 0.15 layers 1-2)
  Top 0.127: IC7.M2 71.61,35.59 72,35.2 73.6,35.2 74,34.8 v74.2,34.8 | IC10.K8 85.2,42.8 v85.2,41.6 A3.TP
  Route2 0.127: v74.2,34.8 81.2,34.8 85.2,38.8 v85.2,41.6
ABUS4  (via drill 0.15 layers 1-2)
  Top 0.127: IC7.M3 70.81,35.59 v71.2,35.2 | IC10.K2 v81.6,42.2 | v81.2,39.6 A4.TP
  Route2 0.127: v81.6,42.2 81.2,41.8 v81.2,39.6 81.2,38.8 80,37.6 76.6,37.6 74.6,35.6 73.8,35.6 73.4,35.2 v71.2,35.2
ABUS5  (via drill 0.15 layers 1-2)
  Top 0.127: IC10.K3 v82.4,41.6 | A5.TP v82,39.6 | IC7.N1 75.21,36.39 v76,35.6
  Route2 0.127: v76,35.6 77.2,36.8 80.4,36.8 82,38.4 v82,39.6 82,41.2 v82.4,41.6
ABUS6  (via drill 0.15 layers 1-2)
  Top 0.127: IC7.N2 71.61,36.39 72,36 v74.4,36 | IC10.J1 80,44 80,42.6 80.8,41.8 v80.8,41.6 A6.TP
  Route2 0.127: v74.4,36 76.4,38 79.8,38 80.8,39 v80.8,41.6
ABUS7  (via drill 0.15 layers 1-2)
  Top 0.127: IC7.N3 70.81,36.39 v71.2,36 | IC10.J2 81.2,44.4 v81.2,42.6 | v80.4,39.6 A7.TP
  Route2 0.127: v71.2,36 73.8,36 76.2,38.4 79.6,38.4 80.4,39.2 v80.4,39.6 80.4,41.8 v81.2,42.6
ABUS8  (via drill 0.15 layers 1-2)
  Top 0.127: IC7.M4 70.01,35.59 v70.4,35.2 | IC10.J3 82,44.4 82,42 v81.6,41.6 A8.TP
  Route2 0.127: v70.4,35.2 70.8,34.8 73.6,34.8 74,35.2 74.8,35.2 76.8,37.2 80.2,37.2 81.6,38.6 v81.6,41.6
ABUS9  (via drill 0.15 layers 1-2)
  Top 0.127: v79.2,41.6 A9.TP | IC10.H1 80.4,45.6 79.2,44.4 v79.2,42.8 | IC7.P1 73.19,37.19 v73.2,37.2
  Route2 0.127: v73.2,37.2 75.6,39.6 79,39.6 79.2,39.8 v79.2,41.6 v79.2,42.8
ABUS10  (via drill 0.15 layers 1-2)
  Top 0.127: IC7.P2 71.61,37.19 72,36.8 75.4,36.8 v76.6,35.6 | IC10.J7 v85.2,44.4 | A10.TP v83.6,41.6
  Route2 0.127: v85.2,44.4 85.2,43.8 83.6,42.2 v83.6,41.6 83.6,38.8 81.2,36.4 77.4,36.4 v76.6,35.6
ABUS11  (via drill 0.15 layers 1-2)
  Top 0.127: IC10.H2 81.2,45.2 80.6,45.2 79.6,44.2 v79.6,42.2 | IC7.P3 70.81,37.19 v71.2,36.8 | v79.6,39.6 A11.TP
  Route2 0.127: v79.6,42.2 v79.6,39.6 79.2,39.2 75.8,39.2 73.4,36.8 v71.2,36.8
ABUS12  (via drill 0.15 layers 1-2)
  Top 0.127: IC7.N4 70.01,36.39 v70.4,36 | IC10.H3 82.8,45.2 v82.8,43.2 | v80,41.6 A12.TP
  Route2 0.127: v70.4,36 70.8,36.4 73.6,36.4 76,38.8 79.4,38.8 80,39.4 v80,41.6 80,42 81.2,43.2 v82.8,43.2
ABUS13  (via drill 0.15 layers 1-2)
  Top 0.127: IC10.H8 v86,45.2 | IC7.R1 73.61,37.99 74.01,37.59 75.81,37.59 77.8,35.6 v78.2,35.6 | A13.TP v84.4,41.6
  Route2 0.127: v86,45.2 85.6,44.8 85.6,43.6 84.4,42.4 v84.4,41.6 84.4,38.8 81.2,35.6 v78.2,35.6
ABUS14  (via drill 0.15 layers 1-2)
  Top 0.127: IC7.R2 71.61,37.99 72,37.6 73.4,37.6 73.8,37.2 75.6,37.2 v77.6,35.2 | IC10.H9 v86.8,45.2 | A14.TP v84.8,39.6
  Route2 0.127: v86.8,45.2 86,44.4 86,43.4 84.8,42.2 v84.8,39.6 84.8,38.8 81.2,35.2 v77.6,35.2
CPU_DDR_DQS0
  Bottom 0.127: R86.1 68.7,46.25 R82.2 C75.1 67.05,46.4 65.8,46.4 65.6,46.2 R26.2
CPU_DDR_DQS1
  Bottom 0.127: R87.1 68.7,47.35 R84.2 C74.1 67.05,47.2 65.8,47.2 64.4,45.8 R31.2
DBUS0  (via drill 0.15 layers 1-2)
  Top 0.127: IC7.U4 70.4,40 70.4,42.2 69.6,43 v69.6,44 | 0.TP v76,49.6 | IC10.A8 v86,50.8
  Route2 0.127: v69.6,44 69.6,44.8 74.4,49.6 v76,49.6 78.4,49.6 79.2,50.4 84,50.4 84.4,50.8 v86,50.8
DBUS1  (via drill 0.15 layers 1-2)
  Top 0.127: IC7.R7 68,38.4 v68,39.2 | 1.TP v78,49.2 | IC10.B7 v84.8,50.4
  Route2 0.127: v68,39.2 68,41.6 70,43.6 70,44.6 74.6,49.2 v78,49.2 78.4,49.2 79.2,50 84,50 84.4,50.4 v84.8,50.4
DBUS2  (via drill 0.15 layers 1-2)
  Top 0.127: IC7.T5 69.19,38.81 v69.6,39.2 | 2.TP v76,48.8 | IC10.B8 v86,50
  Route2 0.127: v69.6,39.2 69.2,39.6 69.2,42.2 70.4,43.4 70.4,44.4 74.8,48.8 v76,48.8 78.4,48.8 79.2,49.6 84,49.6 84.4,50 v86,50
DBUS3  (via drill 0.15 layers 1-2)
  Top 0.127: IC7.U5 v69.6,40 | 3.TP v78,48.4 | IC10.C7 v84.8,49.6
  Route2 0.127: v69.6,40 69.6,42 70.8,43.2 70.8,44.2 75,48.4 v78,48.4 78.4,48.4 79.2,49.2 84,49.2 84.4,49.6 v84.8,49.6
DBUS4  (via drill 0.15 layers 1-2)
  Top 0.127: IC7.V3 70.78,41.38 71.2,41.8 v71.2,43.6 | 4.TP v76,48 | IC10.C8 v86,49.2
  Route2 0.127: v71.2,43.6 71.2,44 75.2,48 v76,48 78.4,48 79.2,48.8 84,48.8 84.4,49.2 v86,49.2
DBUS5  (via drill 0.15 layers 1-2)
  Top 0.127: IC7.V4 69.99,41.19 v70,41.2 | 5.TP v78,47.6 | IC10.D7 v84.8,48.8
  Route2 0.127: v70,41.2 70,41.8 71.6,43.4 71.6,43.8 75.4,47.6 v78,47.6 78.4,47.6 79.2,48.4 84,48.4 84.4,48.8 v84.8,48.8
DBUS6  (via drill 0.15 layers 1-2)
  Top 0.127: IC7.T6 v68.8,39.2 | 6.TP v76,47.2 | IC10.D8 v86,48.4
  Route2 0.127: v68.8,39.2 69.2,38.8 69.8,38.8 70.4,39.4 70.4,41.6 72,43.2 72,43.6 75.6,47.2 v76,47.2 78.4,47.2 79.2,48 84,48 84.4,48.4 v86,48.4
DBUS7  (via drill 0.15 layers 1-2)
  Top 0.127: IC7.R8 v67.2,38.4 | 7.TP v78,46.8 | IC10.E7 v84.8,48
  Route2 0.127: v67.2,38.4 69.8,38.4 70.8,39.4 70.8,41.4 72.4,43 72.4,43.4 75.8,46.8 v78,46.8 78.4,46.8 79.2,47.6 84,47.6 84.4,48 v84.8,48
DBUS8  (via drill 0.15 layers 1-2)
  Top 0.127: IC10.E3 82,48.4 79.8,48.4 78.2,50 v77.4,50 | 8.TP v75.6,50.8 | IC7.V5 69.19,43.59 v69.2,43.6
  Route2 0.127: v77.4,50 76.6,50.8 v75.6,50.8 75,50.8 69.2,45 v69.2,43.6
DBUS9  (via drill 0.15 layers 1-2)
  Top 0.127: IC10.D2 81.2,49.2 80.2,49.2 78.2,51.2 v77.6,51.2 9.TP | IC7.U6 68.39,39.59 68.8,40 v68.8,43.2
  Route2 0.127: v77.6,51.2 74.8,51.2 68.8,45.2 v68.8,43.2
DBUS10  (via drill 0.15 layers 1-2)
  Top 0.127: IC10.D3 83.2,49.6 v83.2,52 | v75.6,51.6 10.TP | IC7.V6 v68.39,42.79 v68.4,42.8
  Route2 0.127: v83.2,52 78.2,52 77.8,51.6 v75.6,51.6 74.6,51.6 68.4,45.4 v68.4,42.8
DBUS11  (via drill 0.15 layers 1-2)
  Top 0.127: IC10.C2 81.2,50 80.6,50 80,50.6 80,51.6 79.6,52 v77.6,52 11.TP | IC7.T7 67.59,38.79 v67.2,39.2
  Route2 0.127: v77.6,52 74.4,52 68,45.6 68,42 67.6,41.6 67.6,39.6 v67.2,39.2
DBUS12  (via drill 0.15 layers 1-2)
  Top 0.127: IC10.C3 82.8,50 v82.8,52.4 | v75.6,52.4 12.TP | IC7.U7 67.59,39.61 v67.2,40
  Route2 0.127: v82.8,52.4 v75.6,52.4 74.2,52.4 67.6,45.8 67.6,42 67.2,41.6 v67.2,40
DBUS13  (via drill 0.15 layers 1-2)
  Top 0.127: IC10.B2 81.2,50.8 v81.2,52.8 | v77.6,52.8 13.TP | IC7.V7 67.59,41.99 v67.2,42.4
  Route2 0.127: v81.2,52.8 v77.6,52.8 74,52.8 67.2,46 v67.2,42.4
DBUS14  (via drill 0.15 layers 1-2)
  Top 0.127: IC10.B3 82,50.8 v82,53.2 | v75.6,53.2 14.TP | IC7.T8 66.8,38.8 v66.4,39.2
  Route2 0.127: v82,53.2 v75.6,53.2 73.8,53.2 66.8,46.2 66.8,39.6 v66.4,39.2
DBUS15  (via drill 0.15 layers 1-2)
  Top 0.127: IC10.A2 v81.6,53.6 | v77.6,53.6 15.TP | IC7.U8 66.8,39.6 v66.4,40
  Route2 0.127: v81.6,53.6 v77.6,53.6 73.6,53.6 66.4,46.4 v66.4,40
DDR_CKE
  Top 0.127: IC10.G1 78.6,44.2 R89.2
DDR_CLK  (via drill 0.15 layers 1-2, 0.15 layers 15-16, 0.25 layers 2-15)
  Top 0.127: v82,46.8 IC10.G2
  Route2 0.127: v82.4,47.2 v82,46.8
  Route15 0.127: v82.8,42 82.8,46.8 v82.4,47.2
  Bottom 0.127: R33.2 77.53,41.8 arc-90 77.79,41.55 arc90 78.04,41.3 78.07,41.3 arc90 78.33,41.55 78.33,42.05 arc-90 78.58,42.3 78.61,42.3 arc-90 78.86,42.05 78.86,41.55 arc90 79.11,41.3 79.15,41.3 arc90 79.4,41.55 79.4,42.05 arc-90 79.65,42.3 79.68,42.3 arc-90 79.94,42.05 79.94,41.55 arc90 80.19,41.3 80.22,41.3 arc90 80.47,41.55 80.47,42.05 arc-90 80.73,42.3 80.76,42.3 arc-90 81.01,42.05 81.01,41.55 arc90 81.26,41.3 81.3,41.3 arc90 81.55,41.55 arc-90 81.8,41.8 82.6,41.8 v82.8,42
DDR_DSQ0  (via drill 0.25)
  Top 0.127: IC10.E8 86,47.6 85,47.6 v84.8,47.4
  Bottom 0.127: v84.8,47.4 84.8,47.2 84,46.4 82.45,46.4 R38.2 82.3,46.25 R83.2
DDR_DSQ1  (via drill 0.25)
  Top 0.127: v83.4,47.2 83,47.6 82,47.6 IC10.E2
  Bottom 0.127: v83.4,47.2 82.45,47.2 R39.2 82.3,47.35 R85.2
DQM0  (via drill 0.15 layers 1-2)
  Top 0.127: RN9.8 v76.6,40.4 | IC10.F8 v86.8,47.6
  Route2 0.127: v76.6,40.4 77,40 77.4,40 78.8,41.4 78.8,43.2 79.2,43.6 84.4,43.6 84.8,44 84.8,44.8 86.8,46.8 v86.8,47.6
DQM1  (via drill 0.15 layers 1-2)
  Top 0.127: RN9.7 76.8,40 v77.2,40.4 | IC10.F2 81.2,46.8 81.2,46.2 81.4,46 82.6,46 83.2,45.4 v83.2,44
  Route2 0.127: v83.2,44 79,44 78.4,43.4 78.4,41.6 v77.2,40.4
DYCS0  (via drill 0.15 layers 1-2)
  Top 0.127: RN10.5 v77,42.2 | v84.4,44.4 IC10.H7
  Route2 0.127: v84.4,44.4 78.8,44.4 78,43.6 78,42.6 77.6,42.2 v77,42.2
EMC_CLK  (via drill 0.15 layers 1-2, 0.15 layers 15-16, 0.25 layers 2-15)
  Top 0.127: IC7.T3 | IC7.T3 v71.2,39.2
  Route2 0.127: v71.2,39.2 71.2,40.6 v72,41.4
  Route15 0.127: v72,41.4 v72,42
  Bottom 0.127: R33.1 72.2,41.8 v72,42
EN_CRS  (via drill 0.15 pad 0.1 layers 1-2, 0.25 layers 2-15, 0.25 pad 0.1)
  Top 0.127: IC7.D18 58.21,29.21 v58.2,29.2
  Route2 0.127: v58.2,29.2 v55.6,29.2
  Route14 0.127: v55.6,29.2 42.8,29.2 v42.4,28.8
  Bottom 0.254: U201.33 42.07,29.13 v42.4,28.8
  Bottom 0.256: R10.1 42.8,28.4 v42.4,28.8
EN_MDC  (via drill 0.15 pad 0.1 layers 1-2, 0.25 layers 2-15, 0.25 pad 0.1)
  Top 0.127: IC7.D9 v65.6,28.8
  Route2 0.127: v65.6,28.8 64,28.8 62.8,27.6 62.8,25.8 61.4,24.4 v55.6,24.4
  Route3 0.127: v46.8,30.8 v46.8,24.4
  Route14 0.127: v46.8,30.8 38.4,30.8 v37.4,31.8 | v55.6,24.4 v46.8,24.4
  Bottom 0.127: U201.25 37.12,31.52 v37.4,31.8
EN_MDIO  (via drill 0.15 pad 0.1 layers 1-2, 0.25 layers 2-15, 0.25 pad 0.1)
  Top 0.127: IC7.C11 64.4,28.4 v64,28
  Route2 0.127: v64,28 63.2,27.2 63.2,25.6 61.6,24 v56,24
  Route3 0.127: v46.4,30.4 v46.4,24
  Route14 0.127: v56,24 v46.4,24 | v46.4,30.4 38,30.4 v36.6,31.8
  Bottom 0.127: U201.24 36.62,31.78 v36.6,31.8
  Bottom 0.15: v36.6,31.8 36.6,32.6 35.72,33.48 34.81,33.48 R68.2
EN_RXCLK  (via drill 0.15 pad 0.1 layers 1-2, 0.25, 0.25 layers 2-15)
  Top 0.127: IC7.E16 v60,29.6
  Route2 0.127: v60,29.6 v56,29.6
  Route3 0.127: v50.4,29.6 v50.4,33.6
  Route14 0.127: v56,29.6 v50.4,29.6 | v50.4,33.6 v42,33.6
  Bottom 0.127: v42,33.6 42,35.6 41.6,36 41.1,36 R40.1
EN_RXD0  (via drill 0.15 pad 0.1 layers 1-2, 0.25, 0.25 layers 2-15)
  Top 0.127: IC7.G15 v60.8,32
  Route2 0.127: v60.8,32 60.4,31.6 v55.6,31.6
  Route3 0.15: v43.2,32 43.2,27.5 v42.4,26.7
  Route14 0.127: v55.6,31.6 44.2,31.6 43.8,32 v43.2,32
  Bottom 0.15: U201.36 41.47,27.63 v42.4,26.7
EN_RXD1  (via drill 0.15 pad 0.1 layers 1-2, 0.25, 0.25 layers 2-15)
  Top 0.127: IC7.F16 60.41,30.81 v60,30.4
  Route2 0.127: v60,30.4 59.6,30 v57.6,30
  Route3 0.127: v41.2,30 v41.2,27
  Route14 0.127: v57.6,30 v41.2,30
  Bottom 0.254: U201.37 41.07,27.13 v41.2,27
EN_RXDV  (via drill 0.15 pad 0.1 layers 1-2, 0.25, 0.25 layers 2-15)
  Top 0.127: IC7.B16 v60,27.2
  Route2 0.127: v60,27.2 v56,27.2
  Route3 0.127: v45.6,27.2 v45.6,29.6
  Route14 0.127: v56,27.2 v45.6,27.2 | v45.6,29.6 v42.4,29.6
  Bottom 0.127: 42.37,29.63 v42.4,29.6
  Bottom 0.254: U201.32 42.37,29.63
  Bottom 0.256: R50.2 42.45,29.65 v42.4,29.6
EN_RXER  (via drill 0.15 pad 0.1 layers 1-2, 0.25 layers 2-15, 0.25 pad 0.1)
  Top 0.127: IC7.D17 v59.2,28.8
  Route2 0.127: v59.2,28.8 v55.2,28.8
  Route14 0.127: v55.2,28.8 43.6,28.8 v42.4,27.6
  Bottom 0.254: U201.34 41.37,28.63 v42.4,27.6
  Bottom 0.256: R11.1 42.85,27.15 v42.4,27.6
EN_TXD0  (via drill 0.15 pad 0.1 layers 1-2, 0.25, 0.25 layers 2-15)
  Top 0.127: IC7.C17 v59.2,28
  Route2 0.127: v59.2,28 v57.2,28
  Route14 0.127: v57.2,28 45,28 42.6,25.6 39.5,25.6 v38,24.1
  Bottom 0.127: U201.4 38.12,24.22 v38,24.1
EN_TXD1  (via drill 0.15 pad 0.1 layers 1-2, 0.25, 0.25 layers 2-15)
  Top 0.127: IC7.C18 58.22,28.42 v58.2,28.4
  Route2 0.127: v58.2,28.4 v56.8,28.4
  Route14 0.127: v56.8,28.4 44.8,28.4 42.4,26 39.25,26 v37.35,24.1
  Bottom 0.127: U201.5 37.62,24.37 v37.35,24.1
EN_TXEN  (via drill 0.15 pad 0.1 layers 1-2, 0.25, 0.25 layers 2-15)
  Top 0.127: IC7.D16 v60,28.8
  Route2 0.127: v60,28.8 59.6,28.4 59.6,27.8 59.4,27.6 v57.6,27.6
  Route14 0.127: v57.6,27.6 45.2,27.6 42.8,25.2 39.75,25.2 v38.65,24.1
  Bottom 0.127: U201.3 38.62,24.13 v38.65,24.1
ETH_SHIELD
  Route3 0.61: ETH.S1 ETH.S2
  Bottom 0.406: R37.2 24.5,12.38 ETH.S1 | RC22.1 37.6,12.56 ETH.S2
  pour Top: 23.2,18.85 39.2,18.85 39.2,0 23.2,0
GND  (via drill 0.15 layers 1-2, 0.15 layers 15-16, 0.25, 0.25 layers 2-15)
  Top 0.127: IC7.P18 IC7.R18 | IC7.P14 | IC7.T15 v61.6,39.2 | IC7.P14 | IC7.P14 v62.4,36.8 | IC7.M12 v63.59,35.59 v63.2,35.2 | IC7.H12 v64,32 | IC7.G12 63.61,31.59 v64,31.2 | IC7.F12 63.61,30.79 v64,30.4 | IC7.F11 64.4,30.8 v64.8,30.4 | IC7.F10 v65.2,30.8 v65.6,30.4 | IC7.G10 v65.6,31.2 | v66.4,31.2 v66.4,31.21 IC7.G8 | IC7.H5 v69.6,32 | IC7.G5 v69.6,31.2 | IC7.F5 v69.6,30.4 | IC7.F6 | IC7.F6 v68,31.2 | IC7.H7 v67.6,32.4 v68,32 | IC7.N5 v68.8,36 IC7.N6 | IC7.M5 v68.8,35.2 | IC7.L5 v68.8,34.4 | IC7.K5 69.19,33.99 v68.8,33.6 | IC7.L7 v67.2,34.4 | v68.8,36.8 IC7.P6 v68,37.6 | IC7.P10 v64.8,37.6 | IC7.P11 v64,37.6 | IC7.P9 v65.6,37.6 | IC7.P8 v66.4,37.6 | IC7.P7 v67.2,37.6 | IC7.R16 v60.8,37.6 | IC7.M10 v65.6,35.2 | IC7.M9 v66.4,35.2 | IC7.L14 v62.4,35.2 | IC7.K13 v63.2,34.4 IC7.K12 | IC10.C1 80.4,49.6 79.6,50.4 79.6,50.6 v79.2,51 | IC10.A1 v80.8,55 | IC10.A3 v82.4,55 | IC10.D9 v88,48.8 | IC10.B9 v88,50.4 | IC10.K1 80.8,43.6 v80.4,43.2 | IC10.F1 79.6,46 v79.2,46 | IC10.E1 80.2,48 79.2,47 v79.2,46.8
  Top 0.15: IC7.R18 58.4,38.4 58,38.4 v57.6,38.8
  Top 0.254: v56,12 56,11.5 | IC11.39 86.37,20.99 IC11.VSSA 90.37,16.99 IC11.21 | C108.2 83.1,14.3 v82.8,14
  Top 0.305: 11,23.73 IC5.10 | IC13.23 56.75,11.25 56.5,11.5 56,11.5 55.5,11.5 55.25,11.25 IC13.17 | IC12.10 11.42,36.5 11.11,36.2 11.11,35.61 | IC11.21 91,16.91 91.1,16.8 v91.1,15.55
  Top 0.406: C64.1 52.1,40.85 C65.1
  Top 0.61: C118.2 7.65,32.5 | 44.07,48.72 C86.2 | 68.77,58.72 C87.2 | 45.34,44.71 C89.2 | 70.04,54.39 C90.2 | R14.1 | 11.11,35.61 IC12.EXP
  Top 1: v84.6,10.6 84.6,13.2 84.55,13.25 83.9,13.25 83.85,13.2 | v81.4,12 81.4,13.45 81.95,14 82.2,14 82.35,14.15 82.55,14.15 82.95,14.55 80.55,14.55 79.5,15.6 | 79.4,17.65 79.5,17.55 80.4,17.55 80.85,18 80.85,18.75 81.05,18.95 81.05,19.7 80.65,20.1 80.65,20.15 80.2,19.7 v79.8,19.7 80,19.7 80,18.4 | C106.1 82.5,23.3 82.5,21.5 83,21.5 83,23.6
  Route2 0.127: v68,32 v67.6,32.4 | v64.4,31.6 v64,32 | v63.8,30.8 63.8,31 v64,31.2 | v65.2,30.8 v64.8,30.4 | v66,30.8 v65.6,30.4 | v66.8,30.8 v66.4,31.2 | v64.2,30 64.2,30.2 v64,30.4 | v67.6,30.8 v67.2,31.2 | v68.4,30.8 v68,31.2 | v65.6,31.8 v65.6,31.2 | v64,37.6 v63.6,38 | v64.4,38 v64.8,37.6 | v65.2,38 v65.6,37.6 | v66,38 v66.4,37.6 | v66.8,38 v67.2,37.6 | v67.6,38 v68,37.6 | v69.2,36.4 v68.8,36.8 | v69.2,35.6 v68.8,36 | v69.2,34.8 v68.8,35.2 | v69.2,34 v68.8,34.4 | v69.2,33.2 v68.8,33.6 | v60.8,37.6 v61.2,38 | v61.6,39.2 v62,38.8 | v62.4,36.8 v62,37.2 | v63.2,35.2 v63.6,35.6 | v65.6,35.2 v65.2,35.6 | v66.4,35.2 v66,35.6 | v62.4,35.2 v62,34.8 | v69.6,32 69.6,31.8 v69.8,31.6 | v69.6,31.2 69.6,31 v69.8,30.8
  Route3 0.127: v68.4,30.8 v67.6,30.8 | v67.6,30.8 v66.8,30.8 v66,30.8 | v66,30.8 v65.2,30.8 64.41,30.8 IC7.F11 | v67.6,32.4 v67.6,30.8 | IC7.F11 64.4,30.2 v64.2,30 | v63.8,30.8 IC7.F11 | v64.4,31.6 IC7.F11 | v66,30.8 66,31.4 v65.6,31.8 | v69.2,33.2 v69.2,34 v69.2,34.8 v69.2,35.6 v69.2,36.4 | v63.6,38 v64.4,38 v65.2,38 v66,38 v66.8,38 v67.6,38
  Bottom 0.254: U201.17 36.62,28.63 | 39.12,29.63 U201.29 | 35.88,26.63 U201.13 | IC9.13 91.75,19.4 C67.2 | IC9.36 91.75,42.56 C68.2 | C105.2 47.94,63.2 BUT2.1 | C104.2 57.71,62.95 BUT1.1 | R4.2 33.95,31.65 v34.4,31.2 | R24.1 v27,50.4
  Bottom 0.305: 36.62,28.63 U201.41 | U201.41 39.12,29.63 | 35.88,26.63 v36,26.75 v36,27.9 v36,29 v37.4,29 v38.75,29 38.49,29 U201.41 | U201.40 39.87,25.63 v38.75,26.75 | C33.2 C32.2 C31.2 | IC8.3 IC8.2 54,44.2 53.8,44.4 53.8,45.2 54.45,45.85 C66.2
  Bottom 0.406: C132.2 v29,28 | IC2.2 IC2.3 37.27,47.84 C1.2 | C21.2 13.77,9.55 DC-IN.1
